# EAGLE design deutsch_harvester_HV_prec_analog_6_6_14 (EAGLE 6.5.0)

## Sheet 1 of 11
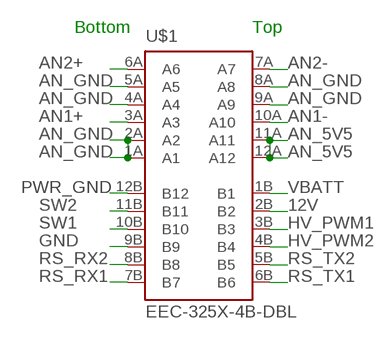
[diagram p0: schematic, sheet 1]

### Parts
U$1  EEC-325X-4B-DBL  [DEUTSCH_EEC_325X-4B]

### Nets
12V: U$1.2B(B2) ; also sheet 2
AN1+: U$1.3A(A3) ; also sheet 7
AN1-: U$1.10A(A10) ; also sheet 7
AN2+: U$1.6A(A6) ; also sheet 9
AN2-: U$1.7A(A7) ; also sheet 9
AN_5V5: U$1.11A(A11) U$1.12A(A12) ; also sheet 3,7,8,9
AN_GND: U$1.1A(A1) U$1.2A(A2) U$1.4A(A4) U$1.5A(A5) U$1.8A(A8) U$1.9A(A9) ; also sheet 7,8,9
GND: U$1.9B(B9) ; also sheet 2,3,4,5,6,8,10,11
HV_PWM1: U$1.3B(B3) ; also sheet 10
HV_PWM2: U$1.4B(B4) ; also sheet 10
PWR_GND: U$1.12B(B12) ; also sheet 2,10
RS_RX1: U$1.7B(B7) ; also sheet 5
RS_RX2: U$1.8B(B8) ; also sheet 5
RS_TX1: U$1.6B(B6) ; also sheet 5
RS_TX2: U$1.5B(B5) ; also sheet 5
SW1: U$1.10B(B10) ; also sheet 4
SW2: U$1.11B(B11) ; also sheet 4
VBATT: U$1.1B(B1) ; also sheet 2

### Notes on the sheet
- Bottom | Top

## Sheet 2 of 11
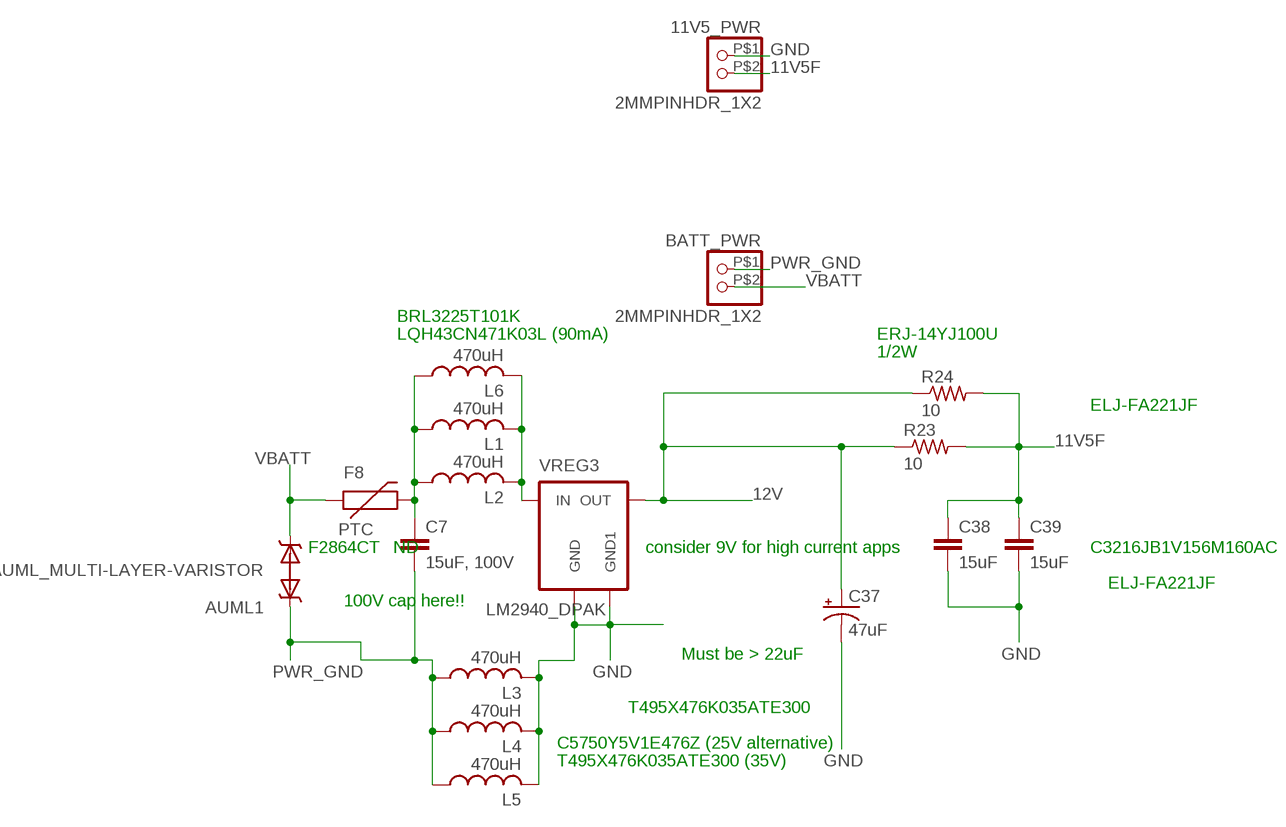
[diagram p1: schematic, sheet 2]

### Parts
11V5_PWR  2MMPINHDR_1X2  [2MMPINHDR_1X2]
AUML1  AUML_MULTI-LAYER-VARISTOR  [SMT_CAP_2220]
BATT_PWR  2MMPINHDR_1X2  [2MMPINHDR_1X2]
C7  15uF, 100V  C-EUC2220K  [C2220K]
C37  47uF  CPOL-USD/7343-31W  [D/7343-31W]
C38  15uF  C-EUC1206  [C1206]
C39  15uF  C-EUC1206  [C1206]
F8  PTC  [R_1206]
L1  470uH  L-USL1812  [L1812]
L2  470uH  L-USL1812  [L1812]
L3  470uH  L-USL1812  [L1812]
L4  470uH  L-USL1812  [L1812]
L5  470uH  L-USL1812  [L1812]
L6  470uH  L-USL1812  [L1812]
R23  10  R-US_R1210  [R1210]
R24  10  R-US_R1210  [R1210]
VREG3  LM2940_DPAK  [DPAK_TO263-3]

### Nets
11V5F: 11V5_PWR.P$2 C38.1 C39.1 R23.2 R24.2 ; also sheet 3
12V: C37.+ R23.1 R24.1 VREG3.3(OUT) ; also sheet 1
GND: 11V5_PWR.P$1 C37.- C38.2 C39.2 L3.2 L4.2 L5.2 VREG3.2(GND) VREG3.4(GND1) ; also sheet 1,3,4,5,6,8,10,11
N$1: C7.1 F8.2 L1.1 L2.1 L6.1
N$3: L1.2 L2.2 L6.2 VREG3.1(IN)
PWR_GND: AUML1.1 BATT_PWR.P$1 C7.2 L3.1 L4.1 L5.1 ; also sheet 1,10
VBATT: AUML1.2 BATT_PWR.P$2 F8.1 ; also sheet 1

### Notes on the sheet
- BRL3225T101K
- LQH43CN471K03L (90mA) | ERJ-14YJ100U
- 1/2W
- ELJ-FA221JF
- F2864CT‑ND | consider 9V for high current apps | C3216JB1V156M160AC
- ELJ-FA221JF
- 100V cap here!!
- Must be > 22uF
- T495X476K035ATE300
- C5750Y5V1E476Z (25V alternative)
- T495X476K035ATE300 (35V)

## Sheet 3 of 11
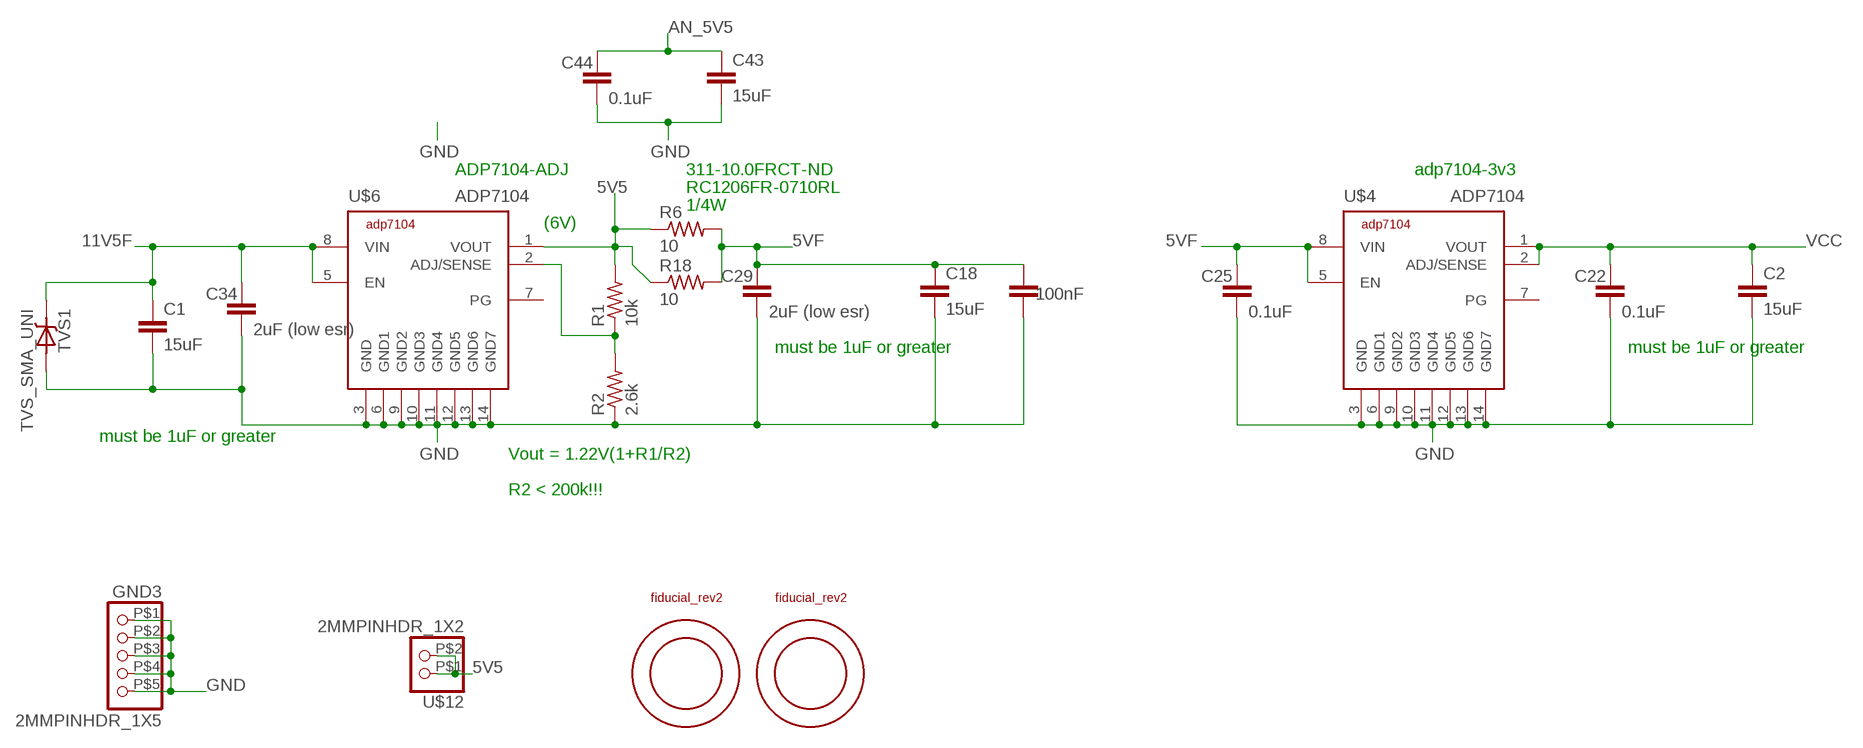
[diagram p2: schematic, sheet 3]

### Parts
C1  15uF  C-EUC1206  [C1206]
C2  15uF  C-EUC1206  [C1206]
C18  15uF  C-EUC1206  [C1206]
C22  0.1uF  C-EUC0805  [C0805]
C23  100nF  C-EUC0805  [C0805]
C25  0.1uF  C-EUC0805  [C0805]
C29  2uF (low esr)  C-EUC0805  [C0805]
C34  2uF (low esr)  C-EUC0805  [C0805]
C43  15uF  C-EUC1206  [C1206]
C44  0.1uF  C-EUC0805  [C0805]
GND3  2MMPINHDR_1X5  [2MMPINHDR_1X5]
R1  10k  R-US_R0805  [R0805]
R2  2.6k  R-US_R0805  [R0805]
R6  10  R-US_R1210  [R1210]
R18  10  R-US_R1210  [R1210]
TVS1  TVS_SMA_UNI  [DO-214AC(SMA)]
U$4  ADP7104  [SO8_GND_PAD]
U$6  ADP7104  [SO8_GND_PAD]
U$10  FIDUCIAL_REV2  [FIDUCIAL_REV2]
U$11  FIDUCIAL_REV2  [FIDUCIAL_REV2]
U$12  2MMPINHDR_1X2  [2MMPINHDR_1X2]

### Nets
5V5: R1.2 R6.1 R18.1 U$6.1(VOUT) U$12.P$1 U$12.P$2 ; also sheet 8
5VF: C18.1 C23.1 C25.1 C29.1 R6.2 R18.2 U$4.5(EN) U$4.8(VIN)
11V5F: C1.1 C34.1 TVS1.C U$6.5(EN) U$6.8(VIN) ; also sheet 2
AN_5V5: C43.1 C44.1 ; also sheet 1,7,8,9
GND: C1.2 C2.2 C18.2 C22.2 C23.2 C25.2 C29.2 C34.2 C43.2 C44.2 GND3.P$1 GND3.P$2 GND3.P$3 GND3.P$4 GND3.P$5 R2.1 TVS1.A U$4.3(GND) U$4.6(GND1) U$4.9(GND2) U$4.10(GND3) U$4.11(GND4) U$4.12(GND5) U$4.13(GND6) U$4.14(GND7) U$6.3(GND) U$6.6(GND1) U$6.9(GND2) U$6.10(GND3) U$6.11(GND4) U$6.12(GND5) U$6.13(GND6) U$6.14(GND7) ; also sheet 1,2,4,5,6,8,10,11
N$6: R1.1 R2.2 U$6.2(ADJ/SENSE)
VCC: C2.1 C22.1 U$4.1(VOUT) U$4.2(ADJ/SENSE) ; also sheet 4,5,6,11
Unconnected: U$4.7(PG) U$6.7(PG)

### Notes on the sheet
- ADP7104-ADJ | 311-10.0FRCT-ND | adp7104-3v3
- RC1206FR-0710RL
- 1/4W
- (6V)
- must be 1uF or greater | must be 1uF or greater
- must be 1uF or greater
- Vout = 1.22V(1+R1/R2)
- R2 < 200k!!!

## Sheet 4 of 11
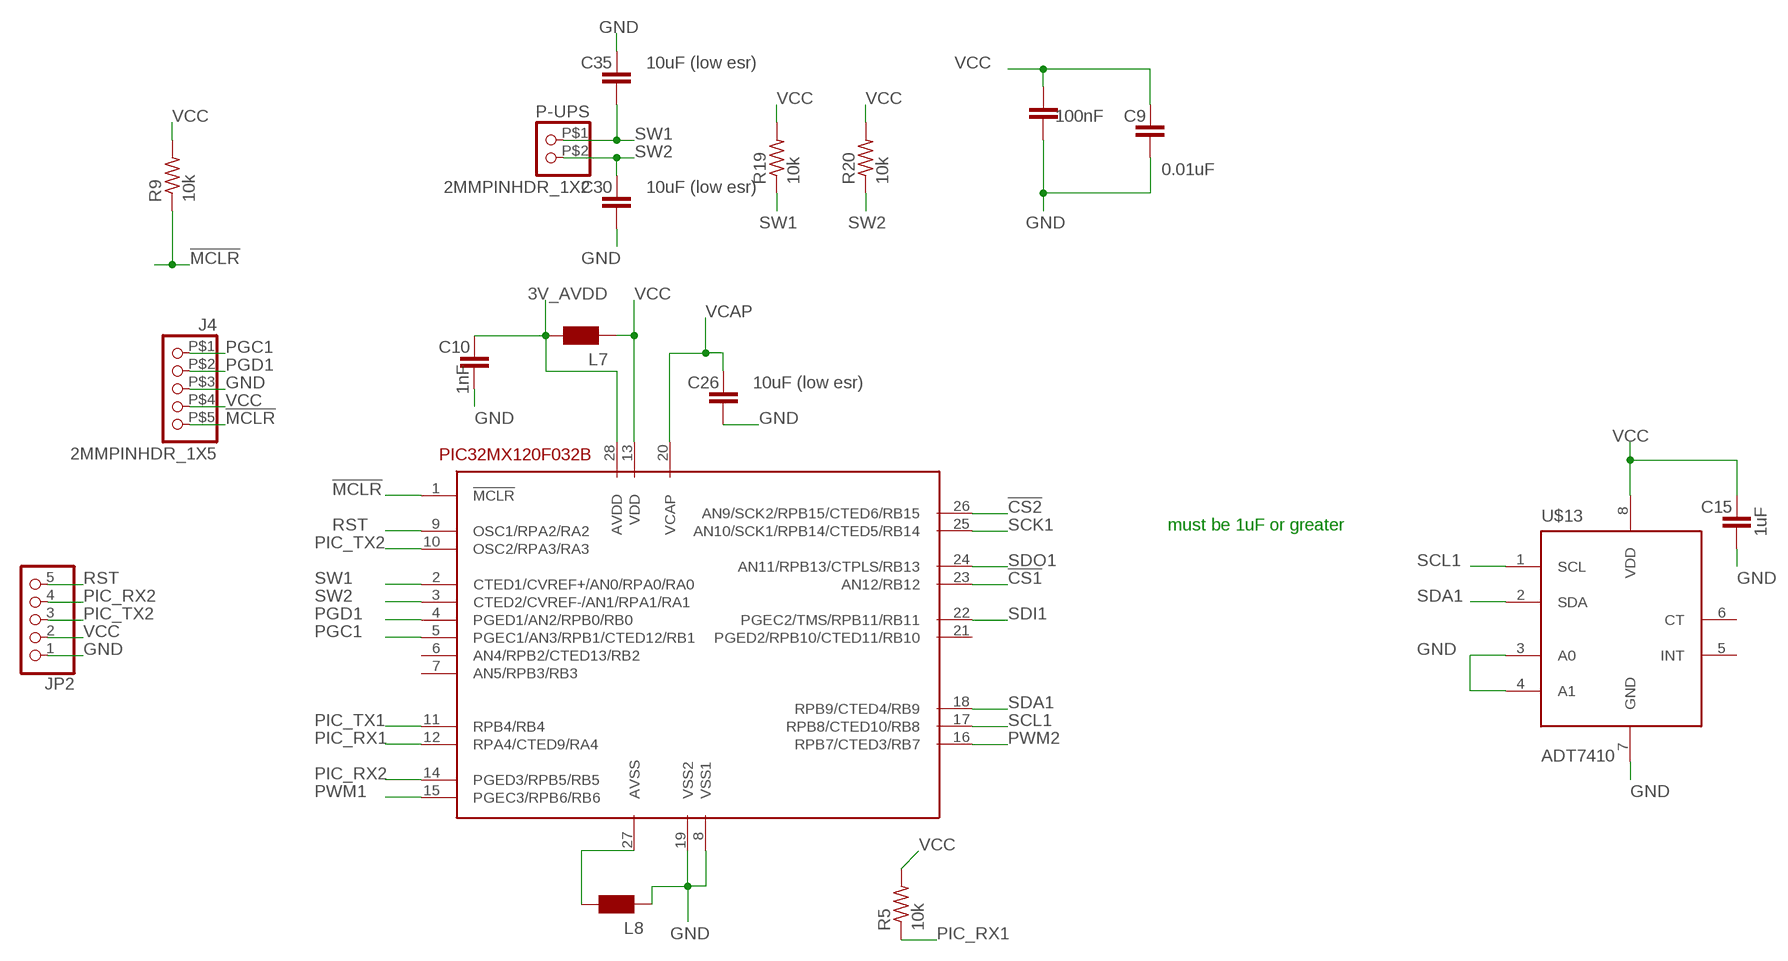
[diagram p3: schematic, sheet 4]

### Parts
C8  100nF  C-EUC0805  [C0805]
C9  0.01uF  C-EUC0805  [C0805]
C10  1nF  C-EUC0805  [C0805]
C15  1uF  C-EUC0805  [C0805]
C26  10uF (low esr)  C-EUC0805  [C0805]
C30  10uF (low esr)  C-EUC0805  [C0805]
C35  10uF (low esr)  C-EUC0805  [C0805]
J4  2MMPINHDR_1X5  [2MMPINHDR_1X5]
JP2  PINHD-1X5  [1X05]
L7  WE-CBF_1206  [1206]
L8  WE-CBF_1206  [1206]
P-UPS  2MMPINHDR_1X2  [2MMPINHDR_1X2]
R5  10k  R-US_R0805  [R0805]
R9  10k  R-US_R0805  [R0805]
R19  10k  R-US_R0805  [R0805]
R20  10k  R-US_R0805  [R0805]
U2  PIC32MX120F032B-28SOIC  [SOICW28_MICROCHIP]
U$13  ADT7410  [SO8]

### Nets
3V_AVDD: C10.1 L7.2 U2.28(AVDD)
!CS1: U2.23(AN12/RB12) ; also sheet 7
!CS2: U2.26(AN9/SCK2/RPB15/CTED6/RB15) ; also sheet 9
!MCLR: J4.P$5 R9.1 U2.1(!MCLR)
GND: C8.2 C9.2 C10.2 C15.2 C26.2 C30.2 C35.1 J4.P$3 JP2.1 L8.1 U2.8(VSS1) U2.19(VSS2) U$13.3(A0) U$13.4(A1) U$13.7(GND) ; also sheet 1,2,3,5,6,8,10,11
N$8: L8.2 U2.27(AVSS)
PGC1: J4.P$1 U2.5(PGEC1/AN3/RPB1/CTED12/RB1)
PGD1: J4.P$2 U2.4(PGED1/AN2/RPB0/RB0)
PIC_RX1: R5.1 U2.12(RPA4/CTED9/RA4) ; also sheet 5
PIC_RX2: JP2.4 U2.14(PGED3/RPB5/RB5) ; also sheet 5
PIC_TX1: U2.11(RPB4/RB4) ; also sheet 5
PIC_TX2: JP2.3 U2.10(OSC2/RPA3/RA3) ; also sheet 5
PWM1: U2.15(PGEC3/RPB6/RB6) ; also sheet 10
PWM2: U2.16(RPB7/CTED3/RB7) ; also sheet 10
RST: JP2.5 U2.9(OSC1/RPA2/RA2)
SCK1: U2.25(AN10/SCK1/RPB14/CTED5/RB14) ; also sheet 7,9
SCL1: U2.17(RPB8/CTED10/RB8) U$13.1(SCL) ; also sheet 6,11
SDA1: U2.18(RPB9/CTED4/RB9) U$13.2(SDA) ; also sheet 6,11
SDI1: U2.22(PGEC2/TMS/RPB11/RB11) ; also sheet 7,9
SDO1: U2.24(AN11/RPB13/CTPLS/RB13)
SW1: C35.2 P-UPS.P$1 R19.1 U2.2(CTED1/CVREF+/AN0/RPA0/RA0) ; also sheet 1
SW2: C30.1 P-UPS.P$2 R20.1 U2.3(CTED2/CVREF-/AN1/RPA1/RA1) ; also sheet 1
VCAP: C26.1 U2.20(VCAP)
VCC: C8.1 C9.1 C15.1 J4.P$4 JP2.2 L7.1 R5.2 R9.2 R19.2 R20.2 U2.13(VDD) U$13.8(VDD) ; also sheet 3,5,6,11
Unconnected: U2.6(AN4/RPB2/CTED13/RB2) U2.7(AN5/RPB3/RB3) U2.21(PGED2/RPB10/CTED11/RB10) U$13.5(INT) U$13.6(CT)

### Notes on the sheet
- must be 1uF or greater

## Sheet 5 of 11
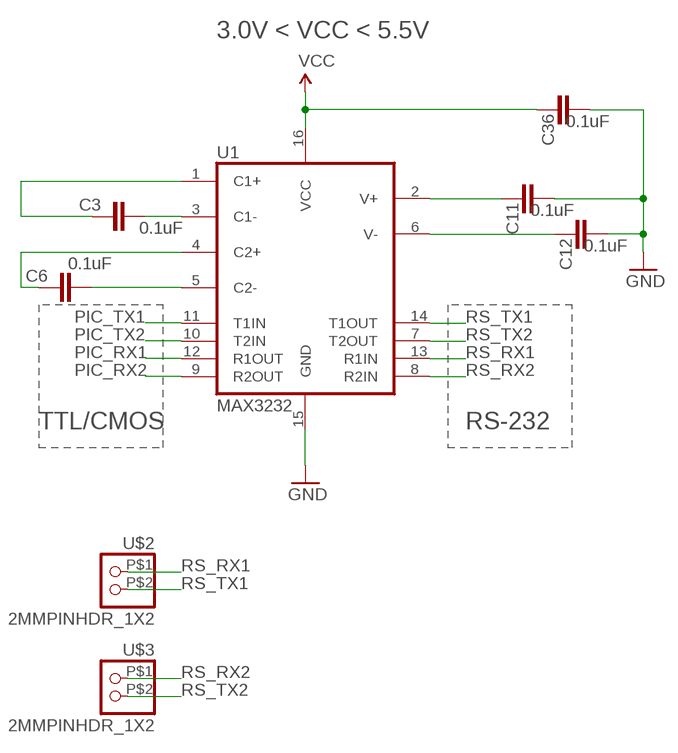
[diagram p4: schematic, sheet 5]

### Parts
C3  0.1uF  C-EUC0805  [C0805]
C6  0.1uF  C-EUC0805  [C0805]
C11  0.1uF  C-EUC0805  [C0805]
C12  0.1uF  C-EUC0805  [C0805]
C36  0.1uF  C-EUC0805  [C0805]
U1  MAX3232  MAX232SOIC16  [SO016]
U$2  2MMPINHDR_1X2  [2MMPINHDR_1X2]
U$3  2MMPINHDR_1X2  [2MMPINHDR_1X2]

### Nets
C1+: C3.1 U1.1(C1+)
C1-: C3.2 U1.3(C1-)
C2+: C6.1 U1.4(C2+)
C2-: C6.2 U1.5(C2-)
GND: C11.2 C12.2 C36.2 U1.15(GND) ; also sheet 1,2,3,4,6,8,10,11
PIC_RX1: U1.12(R1OUT) ; also sheet 4
PIC_RX2: U1.9(R2OUT) ; also sheet 4
PIC_TX1: U1.11(T1IN) ; also sheet 4
PIC_TX2: U1.10(T2IN) ; also sheet 4
RS_RX1: U1.13(R1IN) U$2.P$1 ; also sheet 1
RS_RX2: U1.8(R2IN) U$3.P$1 ; also sheet 1
RS_TX1: U1.14(T1OUT) U$2.P$2 ; also sheet 1
RS_TX2: U1.7(T2OUT) U$3.P$2 ; also sheet 1
V+: C11.1 U1.2(V+)
V-: C12.1 U1.6(V-)
VCC: C36.1 U1.16(VCC) ; also sheet 3,4,6,11

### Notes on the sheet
- 3.0V < VCC < 5.5V
- TTL/CMOS | RS-232

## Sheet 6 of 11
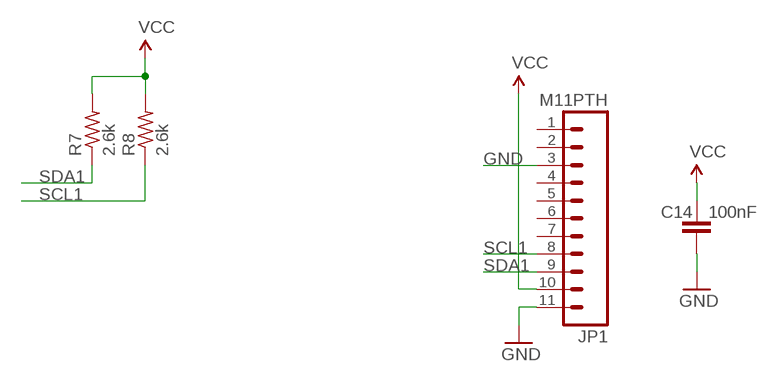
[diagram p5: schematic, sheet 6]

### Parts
C14  100nF  C-EUC0805  [C0805]
JP1  M11PTH  [1X11]
R7  2.6k  R-US_R0805  [R0805]
R8  2.6k  R-US_R0805  [R0805]

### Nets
GND: C14.2 JP1.3 JP1.11 ; also sheet 1,2,3,4,5,8,10,11
SCL1: JP1.8 R8.1 ; also sheet 4,11
SDA1: JP1.9 R7.1 ; also sheet 4,11
VCC: C14.1 JP1.10 R7.2 R8.2 ; also sheet 3,4,5,11
Unconnected: JP1.1 JP1.2 JP1.4 JP1.5 JP1.6 JP1.7

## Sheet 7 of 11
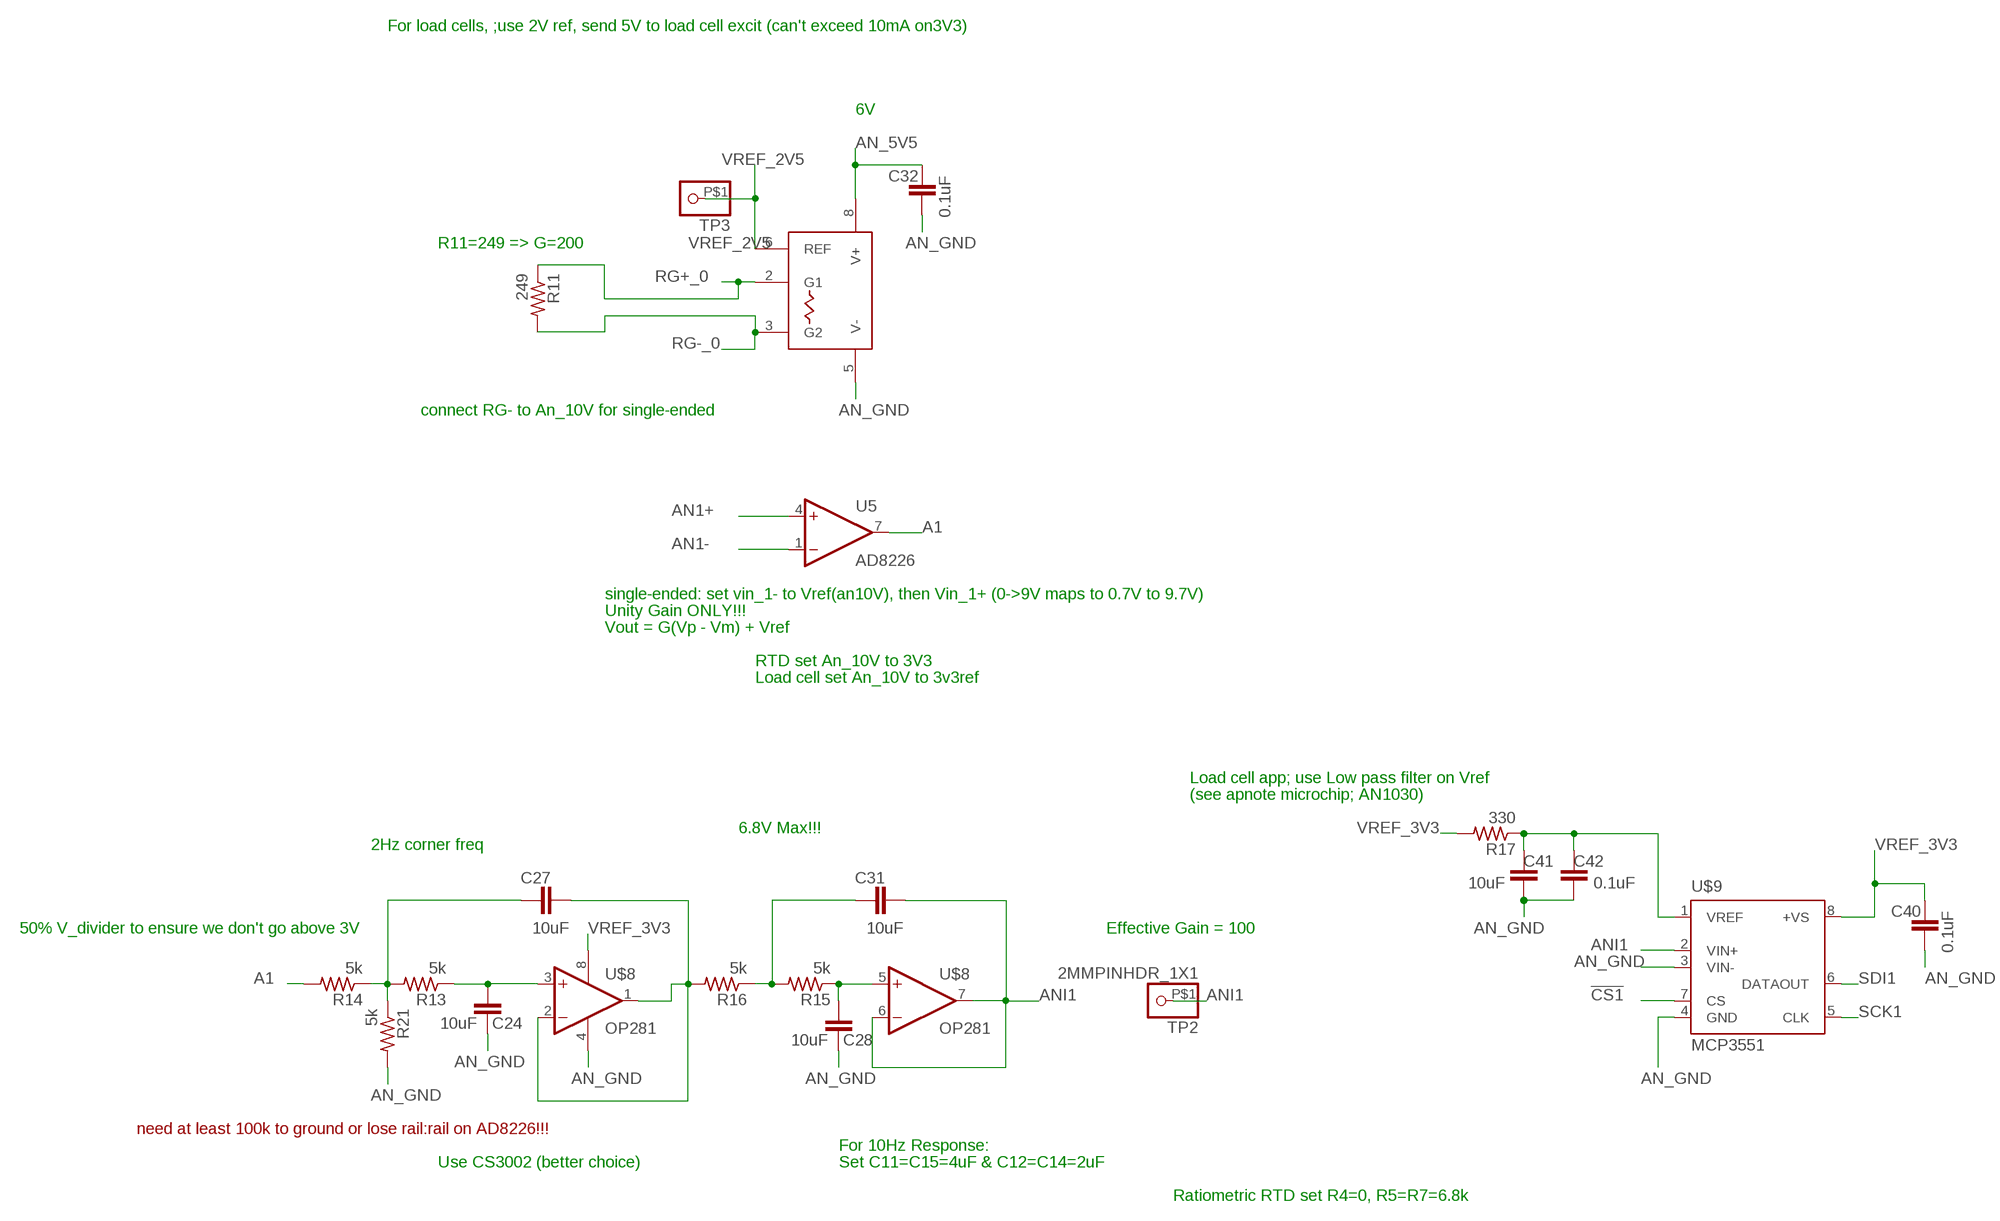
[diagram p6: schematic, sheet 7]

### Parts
C24  10uF  C-EUC0805  [C0805]
C27  10uF  C-EUC0805  [C0805]
C28  10uF  C-EUC0805  [C0805]
C31  10uF  C-EUC0805  [C0805]
C32  0.1uF  C-EUC0805  [C0805]
C40  0.1uF  C-EUC0805  [C0805]
C41  10uF  C-EUC0805  [C0805]
C42  0.1uF  C-EUC0805  [C0805]
R11  249  R-US_R0805  [R0805]
R13  5k  R-US_R0805  [R0805]
R14  5k  R-US_R0805  [R0805]
R15  5k  R-US_R0805  [R0805]
R16  5k  R-US_R0805  [R0805]
R17  330  R-US_R0805  [R0805]
R21  5k  R-US_R0805  [R0805]
TP2  2MMPINHDR_1X1  [2MMPINHDR_1X1]
TP3  2MMPINHDR_1X1  [2MMPINHDR_1X1]
U5  AD8226  [SO8@1]
U$8  OP281  [SO_08]
U$9  MCP3551  [SO_08]

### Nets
!CS1: U$9.7(CS) ; also sheet 4
A1: R14.2 U5.7(OUT)
AN1+: U5.4(+IN) ; also sheet 1
AN1-: U5.1(-IN) ; also sheet 1
AN_5V5: C32.1 U5.8(V+) ; also sheet 1,3,8,9
AN_GND: C24.1 C28.1 C32.2 C40.2 C41.1 C42.1 R21.2 U5.5(V-) U$8.4(V-) U$9.3(VIN-) U$9.4(GND) ; also sheet 1,8,9
ANI1: C31.1 TP2.P$1 U$8.6(-IN2) U$8.7(OUT2) U$9.2(VIN+)
N$2: C24.2 R13.1 U$8.3(+IN1)
N$4: C27.1 R16.2 U$8.1(OUT1) U$8.2(-IN1)
N$5: C27.2 R13.2 R14.1 R21.1
N$9: C41.2 C42.2 R17.1 U$9.1(VREF)
N$13: C31.2 R15.2 R16.1
N$14: C28.2 R15.1 U$8.5(+IN2)
RG+_0: R11.1 U5.2(G1)
RG-_0: R11.2 U5.3(G2)
SCK1: U$9.5(CLK) ; also sheet 4,9
SDI1: U$9.6(DATAOUT) ; also sheet 4,9
VREF_2V5: TP3.P$1 U5.6(REF) ; also sheet 8,9
VREF_3V3: C40.1 R17.2 U$8.8(V+) U$9.8(+VS) ; also sheet 8,9

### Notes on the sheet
- For load cells, ;use 2V ref, send 5V to load cell excit (can't exceed 10mA on3V3)
- 6V
- R11=249 => G=200
- connect RG- to An_10V for single-ended
- single-ended: set vin_1- to Vref(an10V), then Vin_1+ (0->9V maps to 0.7V to 9.7V)
- Unity Gain ONLY!!!
- Vout = G(Vp - Vm) + Vref
- RTD set An_10V to 3V3
- Load cell set An_10V to 3v3ref
- Load cell app; use Low pass filter on Vref
- (see apnote microchip; AN1030)
- 6.8V Max!!!
- 2Hz corner freq
- 50% V_divider to ensure we don't go above 3V | Effective Gain = 100
- need at least 100k to ground or lose rail:rail on AD8226!!!
- For 10Hz Response:
- Use CS3002 (better choice) | Set C11=C15=4uF & C12=C14=2uF
- Ratiometric RTD set R4=0, R5=R7=6.8k

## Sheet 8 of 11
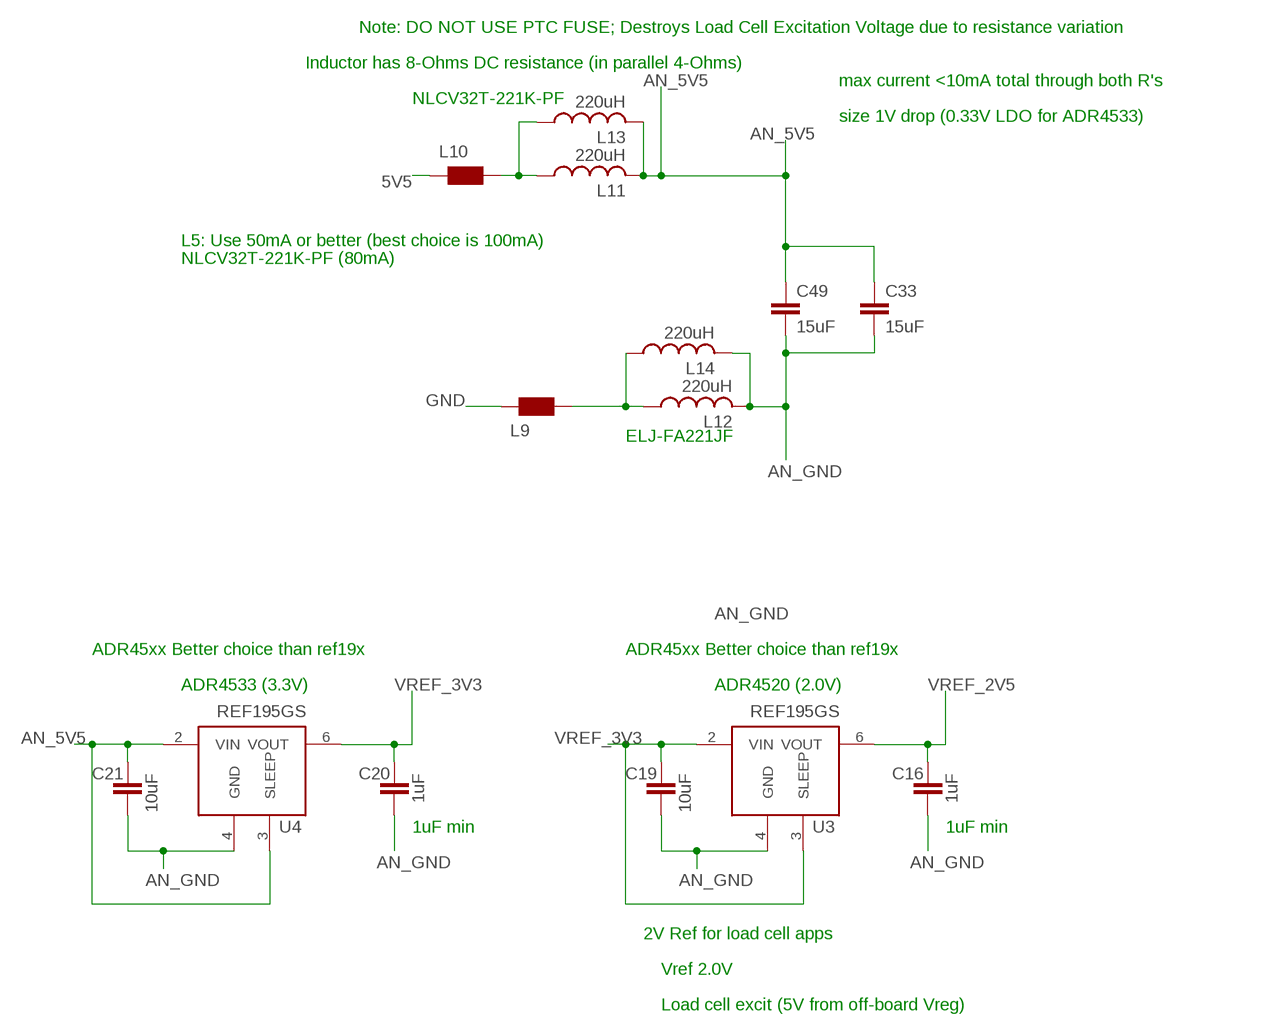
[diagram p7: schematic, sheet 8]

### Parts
C16  1uF  C-EUC0805  [C0805]
C19  10uF  C-EUC0805  [C0805]
C20  1uF  C-EUC0805  [C0805]
C21  10uF  C-EUC0805  [C0805]
C33  15uF  C-EUC1206  [C1206]
C49  15uF  C-EUC1206  [C1206]
L9  WE-CBF_1206  [1206]
L10  WE-CBF_1206  [1206]
L11  220uH  L-USL3225P  [L3225P]
L12  220uH  L-USL3225P  [L3225P]
L13  220uH  L-USL3225P  [L3225P]
L14  220uH  L-USL3225P  [L3225P]
U3  REF195GS  [SO8@1]
U4  REF195GS  [SO8@1]

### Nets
5V5: L10.1 ; also sheet 3
AN_5V5: C21.1 C33.1 C49.1 L11.2 L13.2 U4.2(VIN) U4.3(SLEEP) ; also sheet 1,3,7,9
AN_GND: C16.2 C19.2 C20.2 C21.2 C33.2 C49.2 L12.2 L14.2 U3.4(GND) U4.4(GND) ; also sheet 1,7,9
GND: L9.1 ; also sheet 1,2,3,4,5,6,10,11
N$7: L10.2 L11.1 L13.1
PWR_GND1: L9.2 L12.1 L14.1
VREF_2V5: C16.1 U3.6(VOUT) ; also sheet 7,9
VREF_3V3: C19.1 C20.1 U3.2(VIN) U3.3(SLEEP) U4.6(VOUT) ; also sheet 7,9

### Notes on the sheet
- Note: DO NOT USE PTC FUSE; Destroys Load Cell Excitation Voltage due to resistance variation
- Inductor has 8-Ohms DC resistance (in parallel 4-Ohms)
- max current <10mA total through both R's
- NLCV32T-221K-PF
- size 1V drop (0.33V LDO for ADR4533)
- L5: Use 50mA or better (best choice is 100mA)
- NLCV32T-221K-PF (80mA)
- ELJ-FA221JF
- ADR45xx Better choice than ref19x | ADR45xx Better choice than ref19x
- ADR4533 (3.3V) | ADR4520 (2.0V)
- 1uF min | 1uF min
- 2V Ref for load cell apps
- Vref 2.0V
- Load cell excit (5V from off-board Vreg)

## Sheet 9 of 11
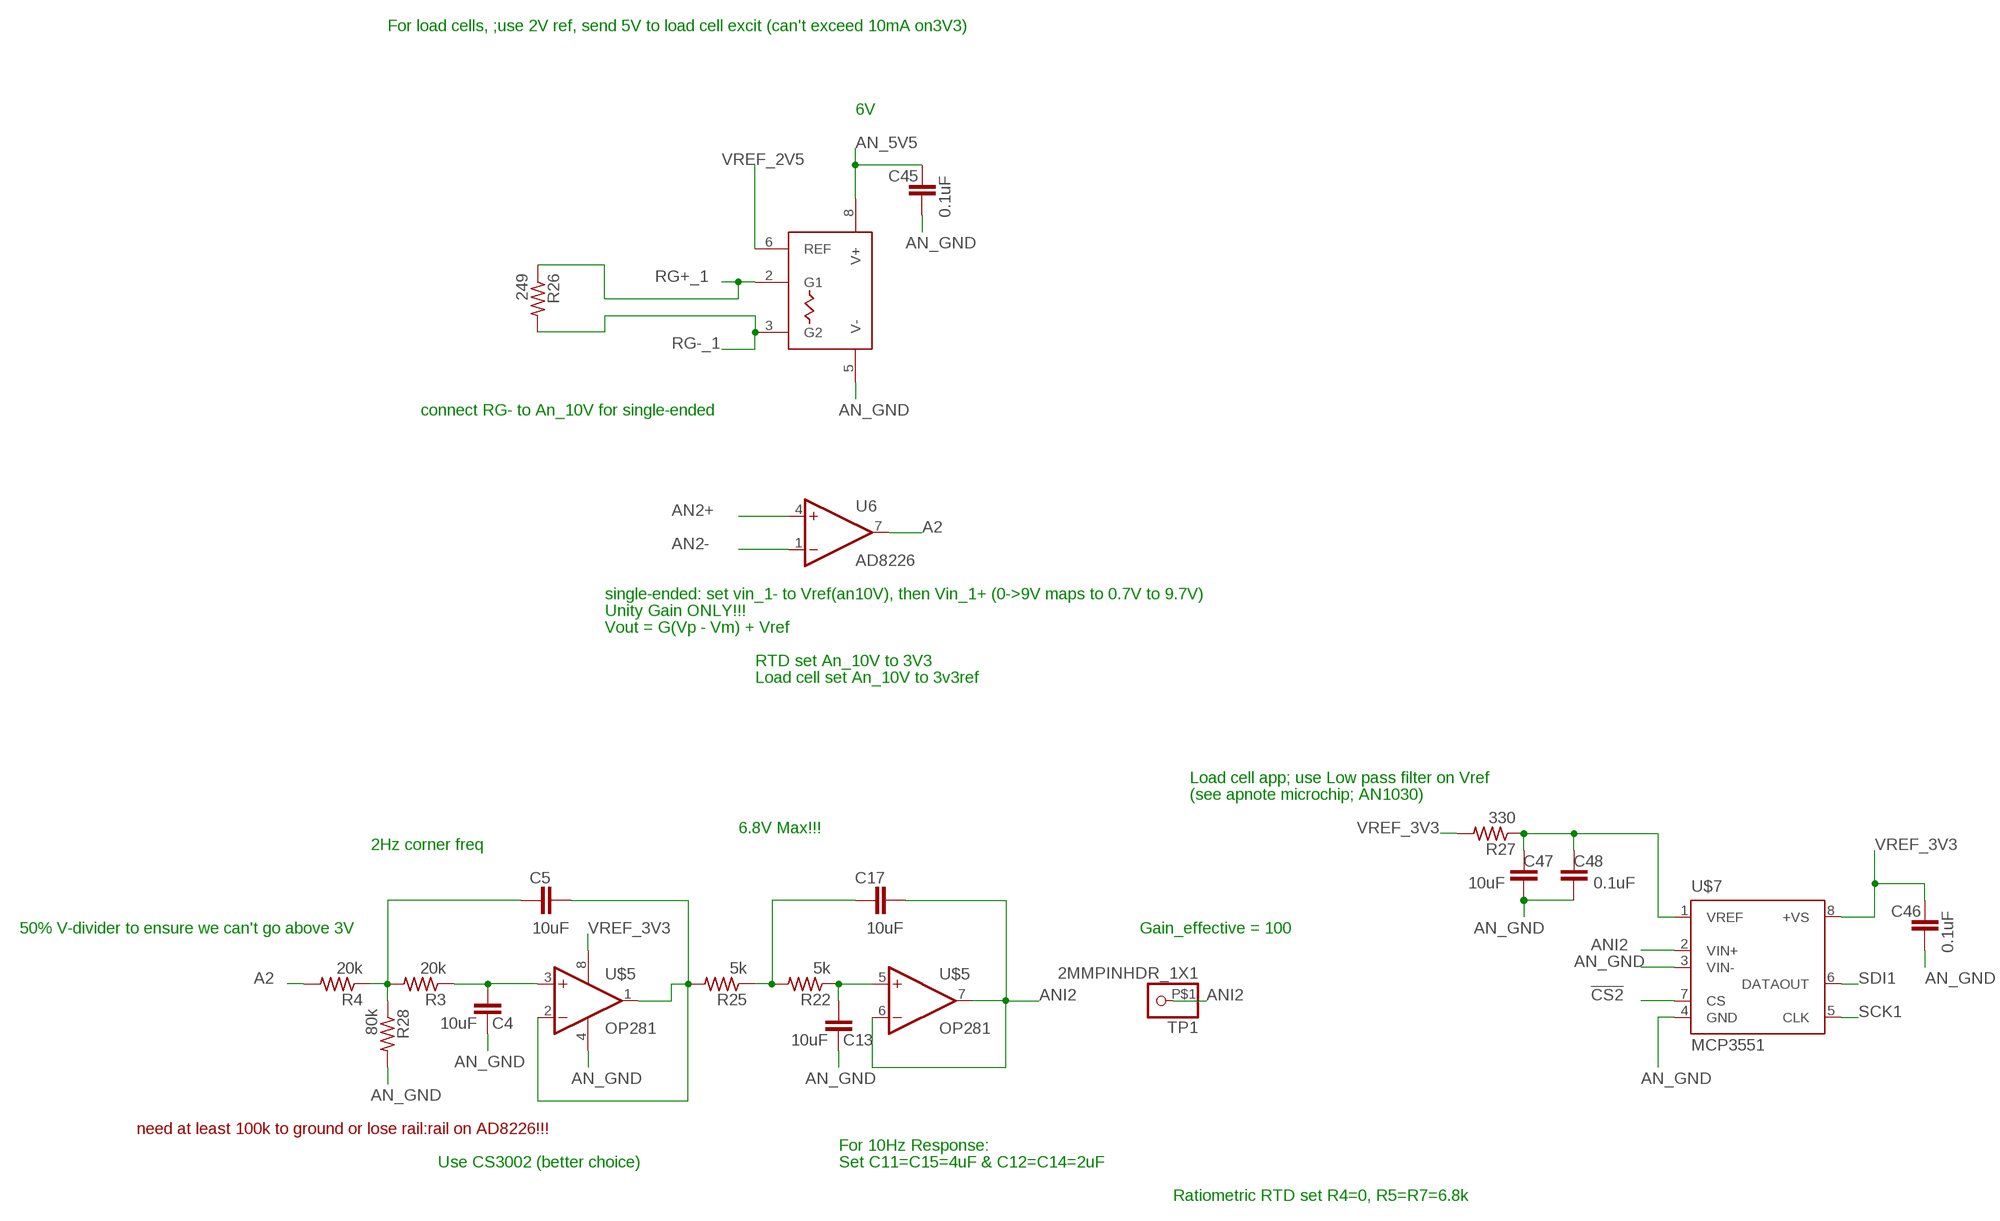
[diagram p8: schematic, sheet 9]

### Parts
C4  10uF  C-EUC0805  [C0805]
C5  10uF  C-EUC0805  [C0805]
C13  10uF  C-EUC0805  [C0805]
C17  10uF  C-EUC0805  [C0805]
C45  0.1uF  C-EUC0805  [C0805]
C46  0.1uF  C-EUC0805  [C0805]
C47  10uF  C-EUC0805  [C0805]
C48  0.1uF  C-EUC0805  [C0805]
R3  20k  R-US_R0805  [R0805]
R4  20k  R-US_R0805  [R0805]
R22  5k  R-US_R0805  [R0805]
R25  5k  R-US_R0805  [R0805]
R26  249  R-US_R0805  [R0805]
R27  330  R-US_R0805  [R0805]
R28  80k  R-US_R0805  [R0805]
TP1  2MMPINHDR_1X1  [2MMPINHDR_1X1]
U6  AD8226  [SO8@1]
U$5  OP281  [SO_08]
U$7  MCP3551  [SO_08]

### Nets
!CS2: U$7.7(CS) ; also sheet 4
A2: R4.2 U6.7(OUT)
AN2+: U6.4(+IN) ; also sheet 1
AN2-: U6.1(-IN) ; also sheet 1
AN_5V5: C45.1 U6.8(V+) ; also sheet 1,3,7,8
AN_GND: C4.1 C13.1 C45.2 C46.2 C47.1 C48.1 R28.2 U6.5(V-) U$5.4(V-) U$7.3(VIN-) U$7.4(GND) ; also sheet 1,7,8
ANI2: C17.1 TP1.P$1 U$5.6(-IN2) U$5.7(OUT2) U$7.2(VIN+)
N$15: C4.2 R3.1 U$5.3(+IN1)
N$16: C5.2 R3.2 R4.1 R28.1
N$17: C17.2 R22.2 R25.1
N$18: C13.2 R22.1 U$5.5(+IN2)
N$19: C5.1 R25.2 U$5.1(OUT1) U$5.2(-IN1)
N$20: C47.2 C48.2 R27.1 U$7.1(VREF)
RG+_1: R26.1 U6.2(G1)
RG-_1: R26.2 U6.3(G2)
SCK1: U$7.5(CLK) ; also sheet 4,7
SDI1: U$7.6(DATAOUT) ; also sheet 4,7
VREF_2V5: U6.6(REF) ; also sheet 7,8
VREF_3V3: C46.1 R27.2 U$5.8(V+) U$7.8(+VS) ; also sheet 7,8

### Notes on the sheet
- For load cells, ;use 2V ref, send 5V to load cell excit (can't exceed 10mA on3V3)
- 6V
- connect RG- to An_10V for single-ended
- single-ended: set vin_1- to Vref(an10V), then Vin_1+ (0->9V maps to 0.7V to 9.7V)
- Unity Gain ONLY!!!
- Vout = G(Vp - Vm) + Vref
- RTD set An_10V to 3V3
- Load cell set An_10V to 3v3ref
- Load cell app; use Low pass filter on Vref
- (see apnote microchip; AN1030)
- 6.8V Max!!!
- 2Hz corner freq
- 50% V-divider to ensure we can't go above 3V | Gain_effective = 100
- need at least 100k to ground or lose rail:rail on AD8226!!!
- For 10Hz Response:
- Use CS3002 (better choice) | Set C11=C15=4uF & C12=C14=2uF
- Ratiometric RTD set R4=0, R5=R7=6.8k

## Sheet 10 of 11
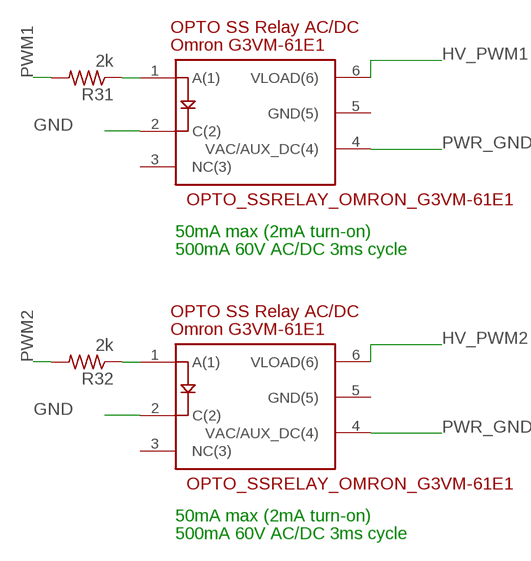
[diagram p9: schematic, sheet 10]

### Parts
R31  2k  R-US_R0805  [R0805]
R32  2k  R-US_R0805  [R0805]
U$43  OPTO_SSRELAY_OMRON_G3VM-61E1  [6-SMD_OMRON_SSRELAY]
U$44  OPTO_SSRELAY_OMRON_G3VM-61E1  [6-SMD_OMRON_SSRELAY]

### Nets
GND: U$43.2(C(2)) U$44.2(C(2)) ; also sheet 1,2,3,4,5,6,8,11
HV_PWM1: U$44.6(VLOAD(6)) ; also sheet 1
HV_PWM2: U$43.6(VLOAD(6)) ; also sheet 1
N$22: R31.1 U$44.1(A(1))
N$23: R32.1 U$43.1(A(1))
PWM1: R31.2 ; also sheet 4
PWM2: R32.2 ; also sheet 4
PWR_GND: U$43.4(VAC/AUX_DC(4)) U$44.4(VAC/AUX_DC(4)) ; also sheet 1,2
Unconnected: U$43.3(NC(3)) U$43.5(GND(5)) U$44.3(NC(3)) U$44.5(GND(5))

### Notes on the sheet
- 50mA max (2mA turn-on)
- 500mA 60V AC/DC 3ms cycle
- 50mA max (2mA turn-on)
- 500mA 60V AC/DC 3ms cycle

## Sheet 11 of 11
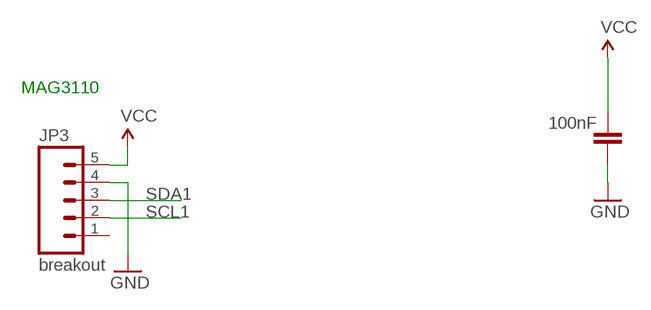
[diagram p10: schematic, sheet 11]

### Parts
C51  100nF  C-EUC0805  [C0805]
JP3  breakout  M05PTH  [1X05]

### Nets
GND: C51.2 JP3.4 ; also sheet 1,2,3,4,5,6,8,10
SCL1: JP3.2 ; also sheet 4,6
SDA1: JP3.3 ; also sheet 4,6
VCC: C51.1 JP3.5 ; also sheet 3,4,5,6
Unconnected: JP3.1

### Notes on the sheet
- MAG3110

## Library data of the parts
11V5_PWR BATT_PWR P-UPS = smd-special_28PIN_PIC32_11_3_2011:2MMPINHDR_1X2
AUML1 = smd-special_28PIN_PIC32_11_3_2011_MOD5_20_13:AUML_MULTI-LAYER-VARISTOR: V18AUMLA2220: 18V cont, 24.5V (5min. jump starts), 25Joule load dump, 40V max Clamp voltage
C1-C36 C38-C49 C51 = rcl:C-EU: CAPACITOR, European symbol
C37 = rcl:CPOL-US: POLARIZED CAPACITOR, American symbol
F8 = smd-special_28PIN_PIC32_11_3_2011_MOD4_1_13:PTC: Little Fuse: 1206L025YR, 16V, 250mA hold, 500mA trip Resetable Fuse
GND3 J4 = smd-special_28PIN_PIC32_11_3_2011_MOD5_20_13:2MMPINHDR_1X5
JP1 = SparkFun-Connectors:M11: Header 11 Standard 11-pin 0.1" header. Use with straight break away headers (SKU : PRT-00116), right angle break away headers (PRT-00553), swiss pins (PRT-00743), machine pins (PRT-00117), and female headers (PRT-00115).
JP2 = pinhead:PINHD-1X5: PIN HEADER
JP3 = SparkFun:M05: Header 5 Standard 5-pin 0.1" header. Use with straight break away headers (SKU : PRT-00116), right angle break away headers (PRT-00553), swiss pins (PRT-00743), machine pins (PRT-00117), and female headers (PRT-00115). Molex polarized connector foot print use with SKU : PRT-08230 with associated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
L1-L6 L11-L14 = rcl:L-US: INDUCTOR, American symbol
L7-L10 = wuerth-elektronik:WE-CBF: SMD EMI Suppression Ferrite Beads
R1-R9 R11 R13-R28 R31 R32 = rcl:R-US_: RESISTOR, American symbol
TP1-TP3 = smd-special_28PIN_PIC32_11_3_2011:2MMPINHDR_1X1
TVS1 = smd-special_28PIN_PIC32_11_3_2011_MOD5_20_13:TVS_SMA_UNI: SMAJ6.0A Uni-directional TVS 6V
U1 = SparkFun-DigitalIC:MAX232: RS232 Transceiver Very common IC. This is generically called 'MAX232', but works with the 3V equivalent MAX3232 generic ICs. Field tested and mother approved. Spark Fun Electronics SKU : COM-00316 (DIP) and COM-00589 (SMD); PROD_ID: IC-08171
U2 = smd-special_28PIN_PIC32_11_3_2011:PIC32MX120F032B-28SOIC
U3 U4 = analog-devices:REF195*: Precision Micropower, Low Dropout, Voltage References Low Supply Current: 45 mikroA max High Output Current: 30 mA Short Circuit Protection
U5 U6 = analog-devices:AD8226: Instrumentation Amp with Over-voltage protection
U$1 = smd-special_28PIN_PIC32_11_3_2011_MOD5_20_13:EEC-325X-4B-DBL
U$2 U$3 U$12 = smd-special_28PIN_PIC32_11_3_2011_MOD5_20_13:2MMPINHDR_1X2
U$4 U$6 = analog-devices:ADP7104: ADP7104 Low Noise LDO Voltage Regulator 15uV noise, 500mA source current
U$5 U$8 = smd-special_28PIN_PIC32_11_3_2011:OP281
U$7 U$9 = smd-special_28PIN_PIC32_11_3_2011:MCP3551
U$10 U$11 = smd-special:FIDUCIAL_REV2
U$13 = analog-devices:ADT7410: Precision I2C Temp Sensor
U$43 U$44 = SparkFun:OPTO_SSRELAY_OMRON_G3VM-61E1
VREG3 = smd-special_28PIN_PIC32_11_3_2011:LM2940_DPAK: lm2940 smt

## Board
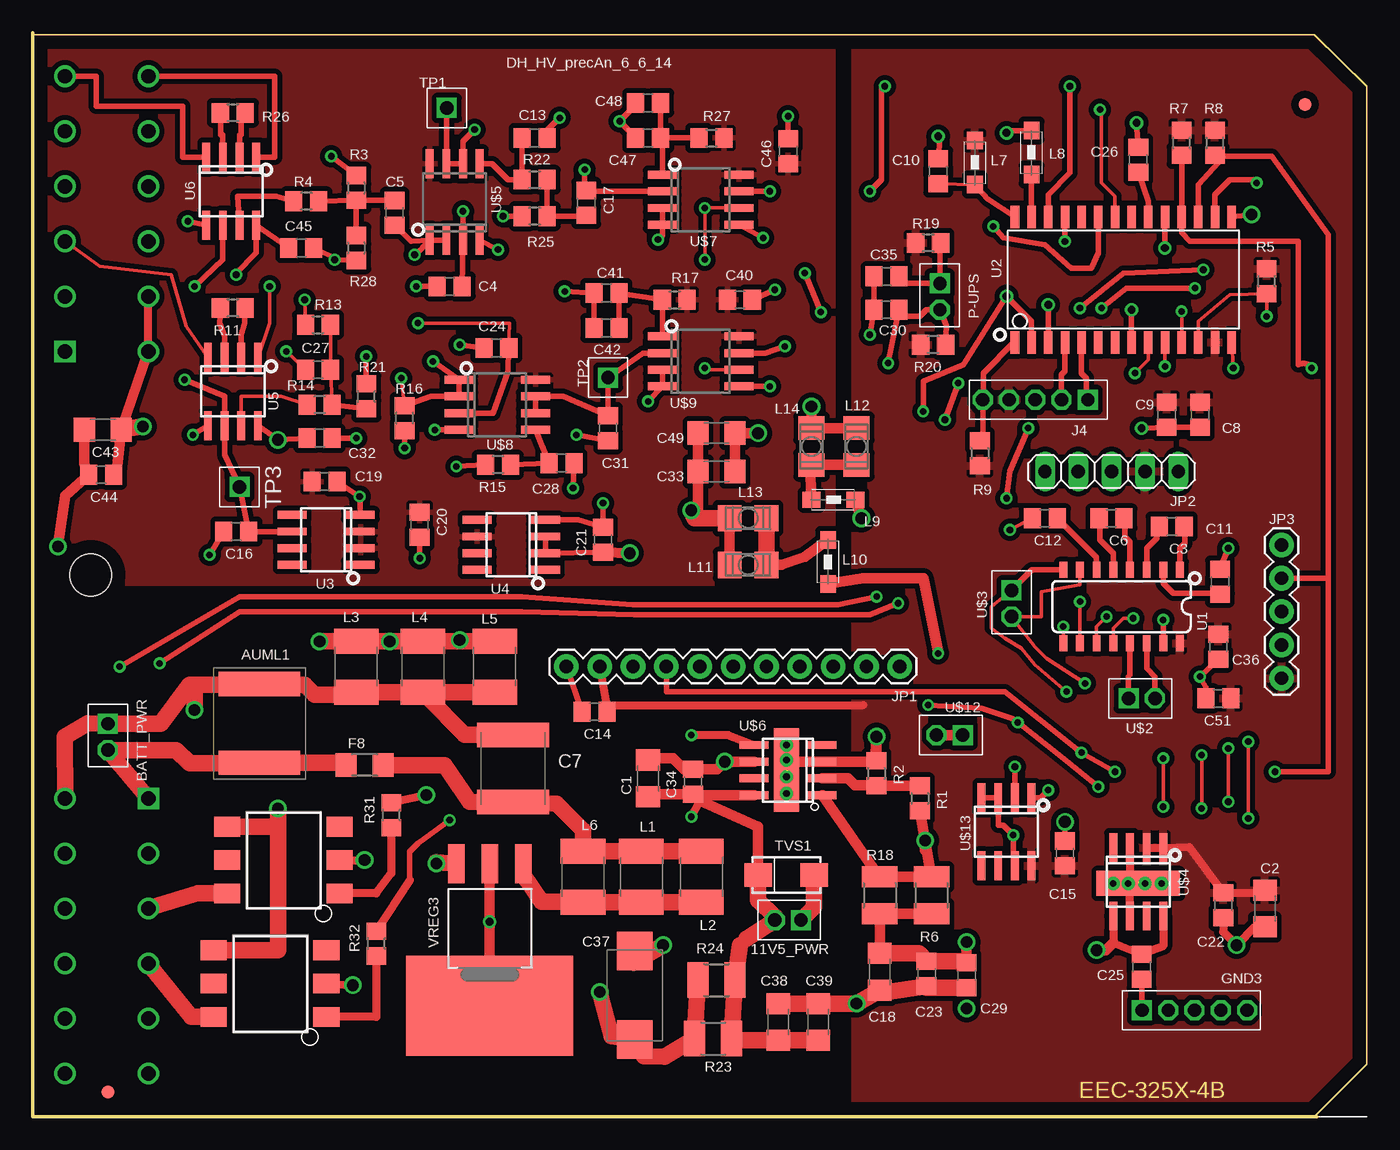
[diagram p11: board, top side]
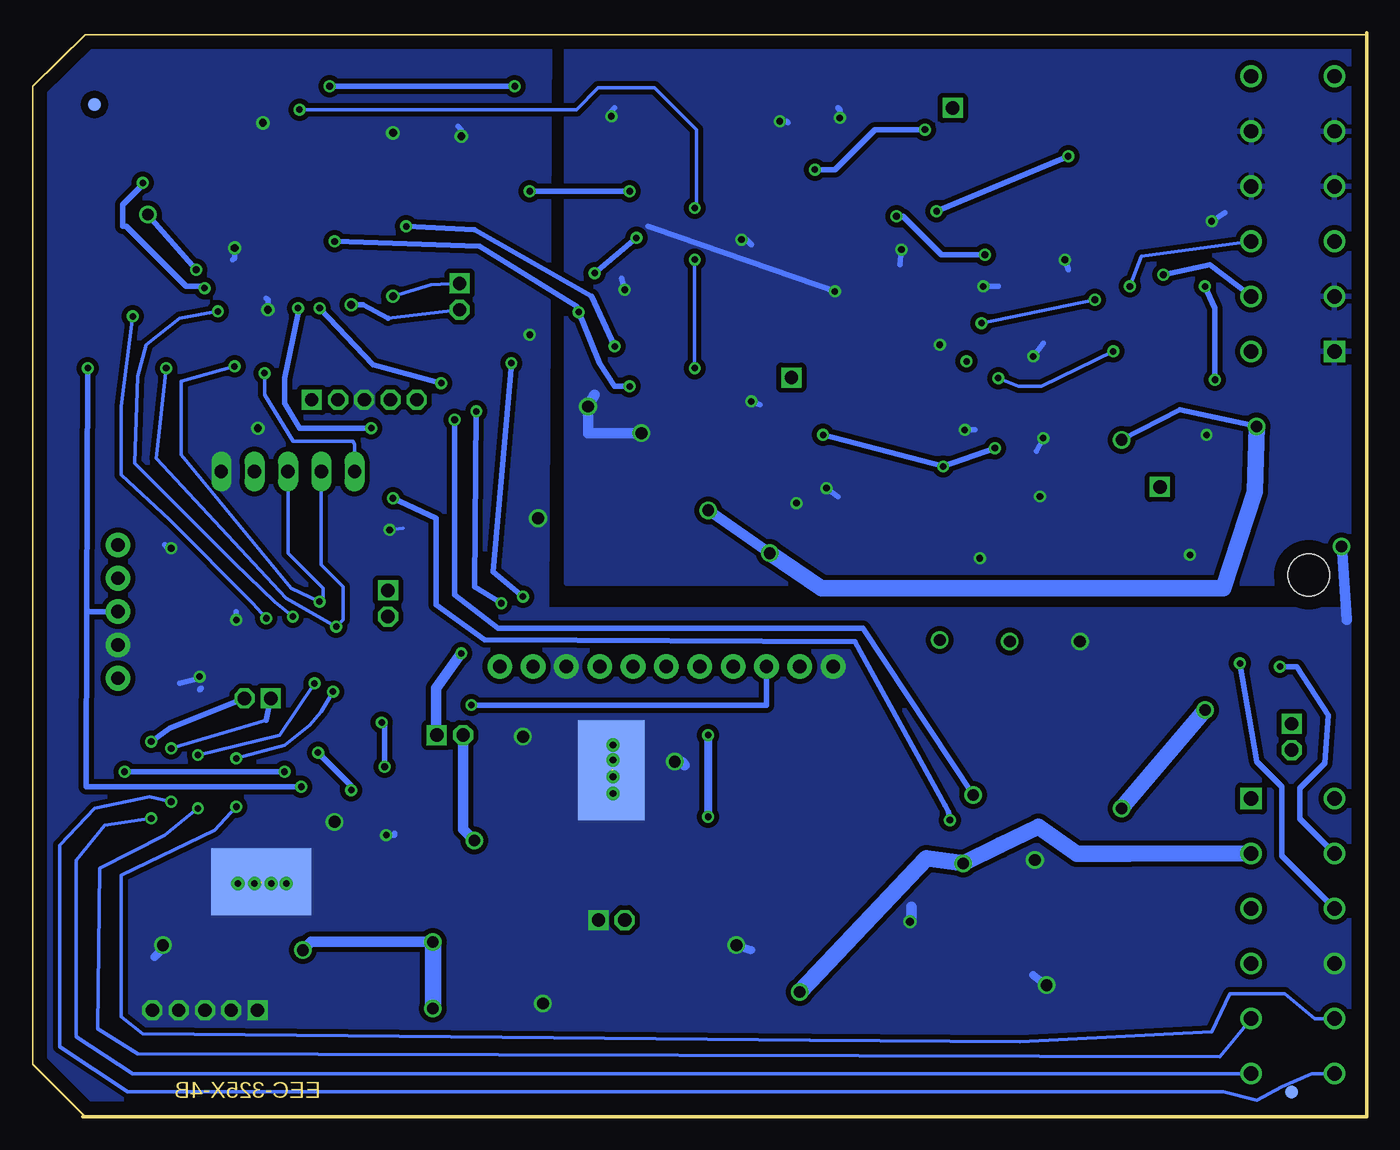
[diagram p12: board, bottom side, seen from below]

Size 101.6 x 82.55 mm. Coordinates in mm from the lower left corner, seen from the top.
Outline: 0,82.55 0,0 97.79,0
Copper layers (1*16): Top 0.035mm / dielectric 1.5mm / Bottom 0.035mm
Design rules "default *": minimum track width 10mil, minimum drill 24mil, track to track 15mil, track to pad 15mil, pad to pad 15mil, via to via 15mil, smd to smd 8mil, copper to edge 40mil, drill to drill 8mil, minimum pad ring 10mil, minimum via ring 8mil, stop-mask expansion 4mil, vias tented up to drill 0mil, thermal gap 10mil

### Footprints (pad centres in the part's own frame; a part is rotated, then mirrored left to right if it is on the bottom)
2MMPINHDR_1X2 = drill 1.016 square: P$1 -1.49,0 | drill 1.016 octagon: P$2 0.51,0
SMT_CAP_2220 = smd 1.85 x 6.2: 1 -3,0; 2 3,0
C1206 = smd 1.6 x 1.8: 1 -1.4,0; 2 1.4,0
C0805 = smd 1.3 x 1.5: 1 -0.95,0; 2 0.95,0
C2220K = smd 1.85 x 5.5: 1 -2.55,0; 2 2.55,0
D/7343-31W = smd 2.95 x 2.7: + 3.375,0; - -3.375,0
R_1206 = smd 1.6 x 1.803: 1 -1.422,0; 2 1.422,0
2MMPINHDR_1X5 = drill 1.016 square: P$1 -0.22,0 | drill 1.016 octagon: P$2 1.78,0; P$3 3.78,0; P$4 5.78,0; P$5 7.78,0
1X11 = drill 1.016 pad 1.88: 1 0,0; 2 2.54,0; 3 5.08,0; 4 7.62,0; 5 10.16,0; 6 12.7,0; 7 15.24,0; 8 17.78,0; 9 20.32,0; 10 22.86,0; 11 25.4,0
1X05 = drill 1.016 long: 1 -5.08,0; 2 -2.54,0; 3 0,0; 4 2.54,0; 5 5.08,0
1X05' = drill 1.016 pad 1.88: 1 0,0; 2 2.54,0; 3 5.08,0; 4 7.62,0; 5 10.16,0
L1812 = smd 1.9 x 3.4: 1 -1.95,0; 2 1.95,0
1206 = smd 1.35 x 1.2: 1 -1.7,0; 2 1.65,0
L3225P = smd 1.8 x 2: 1 -1.4,0; 2 1.4,0
R0805 = smd 1.3 x 1.5: 1 -0.95,0; 2 0.95,0
R1210 = smd 1.6 x 2.7: 1 -1.4,0; 2 1.4,0
2MMPINHDR_1X1 = drill 1.016 square: P$1 0.034,0
DO-214AC(SMA) = smd 2.1 x 1.8: A -2.1,0; C 2.15,0
SO016 = smd 0.6 x 1.2: 1 -4.445,-2.8; 2 -3.175,-2.8; 3 -1.905,-2.8; 4 -0.635,-2.8; 5 0.635,-2.8; 6 1.905,-2.8; 7 3.175,-2.8; 8 4.445,-2.8; 9 4.445,2.8; 10 3.175,2.8; 11 1.905,2.8; 12 0.635,2.8; 13 -0.635,2.8; 14 -1.905,2.8; 15 -3.175,2.8; 16 -4.445,2.8
SOICW28_MICROCHIP = smd 0.65 x 1.7: 1 -7.62,-4.78; 2 -6.35,-4.78; 3 -5.08,-4.78; 4 -3.81,-4.78; 5 -2.54,-4.78; 6 -1.27,-4.78; 7 0,-4.78; 8 1.27,-4.78; 9 2.54,-4.78; 10 3.81,-4.78; 11 5.08,-4.78; 12 6.35,-4.78; 13 7.62,-4.78; 14 8.89,-4.78; 15 8.89,4.78; 16 7.62,4.78; 17 6.35,4.78; 18 5.08,4.78; 19 3.81,4.78; 20 2.54,4.78; 21 1.27,4.78; 22 0,4.78; 23 -1.27,4.78; 24 -2.54,4.78; 25 -3.81,4.78; 26 -5.08,4.78; 27 -6.35,4.78; 28 -7.62,4.78
SO8@1 = smd 0.6 x 2.2: 1 -1.905,-2.6; 2 -0.635,-2.6; 3 0.635,-2.6; 4 1.905,-2.6; 5 1.905,2.6; 6 0.635,2.6; 7 -0.635,2.6; 8 -1.905,2.6
DEUTSCH_EEC_325X-4B = drill 1.1 square: 1A 2.45,58.295; 1B 8.8,24.255 | drill 1.1: 2A 2.45,62.485; 2B 8.8,20.065; 3A 2.45,66.675; 3B 8.8,15.875; 4A 2.45,70.865; 4B 8.8,11.685; 5A 2.45,75.055; 5B 8.8,7.495; 6A 2.45,79.245; 6B 8.8,3.305; 7A 8.8,79.245; 7B 2.45,3.305; 8A 8.8,75.055; 8B 2.45,7.495; 9A 8.8,70.865; 9B 2.45,11.685; 10A 8.8,66.675; 10B 2.45,15.875; 11A 8.8,62.485; 11B 2.45,20.065; 12A 8.8,58.295; 12B 2.45,24.255 | hole 3.2: 4.41,41.28
SO8_GND_PAD = smd 0.6 x 2.2: 1 -2.032,-2.727; 2 -0.762,-2.727; 3 0.508,-2.727; 4 1.778,-2.727; 5 1.778,2.473; 6 0.508,2.473; 7 -0.762,2.473; 8 -2.032,2.473 | smd 6.35 x 1.905: 9 -0.127,0 | smd 7.62 x 5.08 bottom: 10 -0.127,-0.127 | drill 0.5: 11 -1.905,0; 12 -0.635,0; 13 0.635,0; 14 1.778,0
SO_08 = smd 0.6 x 2.2: 1 -1.905,-2.6; 2 -0.635,-2.6; 3 0.635,-2.6; 4 1.905,-2.6; 5 1.905,3.235; 6 0.635,3.235; 7 -0.635,3.235; 8 -1.905,3.235
FIDUCIAL_REV2 = smd 1 x 1: 1 0,0 | smd 1 x 1 bottom: 2 0,0
SO8 = smd 0.6 x 2.2: 1 -1.905,-2.6; 2 -0.635,-2.6; 3 0.635,-2.6; 4 1.905,-2.6; 5 1.905,2.6; 6 0.635,2.6; 7 -0.635,2.6; 8 -1.905,2.6
6-SMD_OMRON_SSRELAY = smd 1.5 x 2: 1 -3.81,-5.08; 2 -1.27,-5.08; 3 1.27,-5.08; 4 1.27,3.493; 5 -1.27,3.493; 6 -3.81,3.493
DPAK_TO263-3 = smd 1.27 x 2.997: 1 -2.553,-4.928; 2 -0.013,-4.928; 3 2.527,-4.928 | smd 12.7 x 7.62: 4 0,5.893

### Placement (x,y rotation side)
11V5_PWR  57.02,14.99 180 top
AUML1  17.27,29.97 270 top
BATT_PWR  5.71,28.45 270 top
C1  46.86,25.78 90 top
C2  93.85,15.88 270 top
C3  86.74,44.96 180 top
C4  31.75,63.25 0 top
C5  27.56,68.83 90 top
C6  82.17,45.59 180 top
C7  36.58,26.54 90 top
C8  88.9,53.47 270 top
C9  86.36,53.47 270 top
C10  68.96,72.01 90 top
C11  90.42,40.77 90 top
C12  77.09,45.59 180 top
C13  38.23,74.55 180 top
C14  42.8,30.86 180 top
C15  78.61,20.07 90 top
C16  15.49,44.58 180 top
C17  42.16,69.6 270 top
C18  64.52,11.05 270 top
C19  22.23,48.39 0 top
C20  29.46,45.09 270 top
C21  43.43,43.94 90 top
C22  90.68,16.13 270 top
C23  68.07,10.92 270 top
C24  35.31,58.55 0 top
C25  84.45,11.43 270 top
C26  84.2,72.9 90 top
C27  21.72,56.9 0 top
C28  40.26,49.78 180 top
C29  71.12,10.79 270 top
C30  65.02,61.47 180 top
C31  43.81,52.45 270 top
C32  21.84,51.69 0 top
C33  52.07,49.15 0 top
C34  50.29,25.53 90 top
C35  65.02,64.01 0 top
C36  90.3,35.81 270 top
C37  45.85,9.27 270 top
C38  56.77,7.24 90 top
C39  59.82,7.24 90 top
C40  53.85,62.23 0 top
C41  43.69,62.74 0 top
C42  43.69,60.07 0 top
C43  5.33,52.32 180 top
C44  5.21,48.9 180 top
C45  20.45,66.17 0 top
C46  57.53,73.53 90 top
C47  46.86,74.55 0 top
C48  46.86,77.22 0 top
C49  52.07,52.07 0 top
C51  90.3,31.88 180 top
F8  25.27,26.8 0 top
GND3  84.71,8.13 0 top
J4  80.14,54.61 180 top
JP1  66.04,34.29 180 top
JP2  82.17,49.15 180 top
JP3  breakout  [1X05']  95.12,43.56 270 top
L1  46.35,18.29 270 top
L2  50.93,18.29 270 top
L3  24.64,34.29 90 top
L4  29.72,34.29 90 top
L5  35.18,34.29 90 top
L6  41.91,18.29 270 top
L7  71.75,72.64 270 top
L8  76.07,73.41 270 top
L9  60.96,46.99 180 top
L10  60.58,42.29 90 top
L11  54.48,42.04 180 top
L12  62.74,51.05 90 top
L13  54.48,45.59 180 top
L14  59.31,51.05 90 top
P-UPS  69.09,61.98 270 top
R1  67.56,24.26 270 top
R2  64.26,26.16 270 top
R3  24.64,70.74 270 top
R4  20.83,69.72 180 top
R5  93.98,63.63 90 top
R6  68.45,16.89 270 top
R7  87.5,74.17 90 top
R8  90.04,74.17 90 top
R9  72.14,50.55 270 top
R11  15.24,61.59 180 top
R13  21.72,60.33 0 top
R14  21.84,54.23 180 top
R15  35.43,49.66 180 top
R16  28.32,53.21 90 top
R17  48.9,62.23 0 top
R18  64.52,16.89 270 top
R19  68.2,66.55 180 top
R20  68.58,58.8 180 top
R21  25.4,54.86 90 top
R22  38.23,71.37 0 top
R23  51.82,5.97 0 top
R24  52.07,10.41 0 top
R25  38.23,68.58 180 top
R26  15.24,76.45 180 top
R27  51.69,74.55 0 top
R28  24.64,66.17 270 top
R31  27.3,22.99 90 top
R32  26.16,13.21 90 top
TP1  31.5,76.83 0 top
TP2  43.81,56.26 90 top
TP3  15.75,48.01 270 top
TVS1  57.4,18.41 180 top
U1  82.93,38.86 180 top
U2  82.42,63.75 0 top
U3  22.35,43.94 90 top
U4  36.45,43.56 90 top
U5  15.24,55.24 180 top
U6  15.11,70.48 180 top
U$1  0,0 0 top
U$2  84.96,31.88 0 top
U$3  74.55,38.61 270 top
U$4  84.07,17.78 180 top
U$5  32.13,69.34 0 top
U$6  57.4,26.54 90 top
U$7  50.55,69.85 270 top
U$8  35.05,54.23 270 top
U$9  50.55,57.53 270 top
U$10  5.71,1.91 0 top
U$11  96.9,77.09 0 top
U$12  69.34,29.08 180 top
U$13  74.17,21.72 180 top
U$43  17.27,11.43 90 top
U$44  18.29,20.83 90 top
VREG3  34.8,14.35 180 top

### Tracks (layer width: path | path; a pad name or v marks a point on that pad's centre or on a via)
3V_AVDD
  Top 0.254: C10.1 L7.2
  Top 0.406: U2.28 72.72,69.93 L7.2
5V5  (via drill 0.5, 0.89)
  Top 0.813: U$6.1 64.32,18.48 R18.1 R6.1 v67.96,21.05 | R1.2 v67.96,21.05 | U$12.P$2 U$12.P$1 | v68.96,35.31 67.82,41.02 63.25,41.02 L10.1 | v67.96,21.05 67.96,20.32 68.12,20.16
  Bottom 0.813: 70.96,29.08 U$12.P$1 70.87,30.19 70.87,32.64 v68.96,35.31 | U$12.P$2 68.83,21.92 v67.96,21.05
5VF  (via drill 0.89)
  Top 0.61: U$4.8 86.11,13.02 C25.1 82.3,13.27 U$4.5
  Top 0.813: R6.2 R18.2 C18.1 | 70.99,11.87 C29.1 v71.12,13.34 | v81.03,12.7 81.73,12.7 82.3,13.27
  Top 1.27: C18.1 67.5,12.45 C23.1 70.99,11.87
  Bottom 0.813: v71.12,13.34 80.39,13.34 v81.03,12.7
  Bottom 1.27: v71.12,13.34 v71.12,8.26
11V5F  (via drill 0.51)
  Top 0.61: C38.1 | U$6.5 52.96,29.08 v50.16,29.08 | v50.16,22.86 50.81,24.06
  Top 0.813: 54.35,13.58 53.85,13.07 | 11V5_PWR.P$2 56.51,15.24 | TVS1.C 55.24,22.1 50.81,24.06 C34.1 | C34.1 47.06,24.58 C1.1 | U$6.8 50.36,24.51 C34.1
  Top 1.27: 53.85,13.07 R24.2 R23.2 53.85,5.84 C38.1 | 11V5_PWR.P$2 54.35,13.58 | 56.51,15.24 55.24,16.51 TVS1.C | C38.1 C39.1
  Bottom 0.61: v50.16,29.08 v50.16,22.86
12V  (via drill 0.89)
  Top 0.813: 50.29,5.84 R23.1
  Top 1.27: 32.26,19.79 VREG3.3 30.73,19.41 v30.73,19.3 | R24.1 R23.1 48.13,4.57 46.54,4.63 C37.+ 44.07,6.15 v43.18,9.53
  Bottom 1.27: v43.18,9.53 33.53,19.68 v30.73,19.3 27.94,20.68 25.02,22.1 22.07,20.04 18.09,20.04 U$1.2B
!CS1  (via drill 0.5)
  Top 0.406: U$9.7 55.75,58.17 v57.28,58.67 | v73.15,67.82 73.91,66.93 77.09,66.42 79.12,64.64 80.64,64.64 81.15,65.79 U2.23
  Bottom 0.406: v57.28,58.67 59.05,62.48 67.94,67.56 v73.15,67.82
!CS2  (via drill 0.51)
  Top 0.406: U$7.7 v56.13,70.48 | v63.75,70.48 64.64,71.37 64.64,78.23 v64.9,78.49 | v78.99,78.49 78.99,71.88 77.34,70.23 U2.26
  Bottom 0.406: v56.13,70.48 v63.75,70.48 | v64.9,78.49 v78.99,78.49
!MCLR
  Top 0.406: U2.1 74.72,58.97 72.39,56.64 72.39,54.64 J4.P$5 72.36,51.59 R9.1
A1
  Top 0.254: U5.7 15.88,54.86 18.92,54.86 R14.2
A2
  Top 0.406: U6.7 15.62,70.1 18.54,70.1 R4.2
AN1+
  Top 0.254: U5.4 11.68,60.2 10.54,64.14 5.08,64.77 U$1.3A
AN1-  (via drill 0.51)
  Top 0.254: U5.1 18.03,60.45 v18.03,63.25
  Bottom 0.254: v18.03,63.25 17.14,65.53 U$1.10A
AN2+
  Top 0.406: U6.4 11.43,73.08 11.43,76.96 4.83,76.96 4.83,79.25 U$1.6A
AN2-
  Top 0.406: U6.1 18.41,73.08 18.41,79.25 U$1.7A
AN_5V5  (via drill 0.51, 0.89)
  Top 0.406: C21.1 U4.2 U4.3 | v15.49,64.14 15.49,64.26 17.02,65.79 U6.8 C45.1 | U5.8 v18.67,51.56 C32.1
  Top 0.61: U$1.12A U$1.11A
  Top 0.813: L11.2 L13.2 | U$1.11A | C44.1 6.35,48.84 C43.1 U$1.12A | C21.1 v45.47,42.93 | 50.55,45.59 v50.15,46.2 50.67,46.2 C33.1 C49.1
  Top 1.27: v8.38,52.58 C43.1 | L13.2 50.55,45.59 50.42,45.59 v50.15,46.2
  Bottom 0.406: v15.49,64.14 11.94,64.9 U$1.11A | v18.67,51.56 14.22,53.85 v8.38,52.58
  Bottom 0.813: v45.47,42.93 v50.15,46.2
  Bottom 1.27: v45.47,42.93 41.53,40.26 10.92,40.26 8.51,47.62 v8.38,52.58
AN_GND  (via drill 0.5, 0.51, 0.9)
  Top 0.406: v43.43,46.74 C21.2 41.53,45.47 U4.4 | C20.2 v29.46,42.55 | C19.2 v24.89,47.24 U3.4 | C16.2 v13.46,42.8 | U5.5 v12.19,51.94 | C24.1 v32.51,58.8 | U$9.3 U$9.4 v46.86,54.48 | v40.51,62.87 C41.1 C42.1 | C28.1 v41.15,47.88 | U$8.4 v30.61,52.32 | R21.2 v25.4,57.91 | C32.2 v24.64,51.69 | C40.2 v56.52,62.99 | C4.1 v29.21,63.25 | U$5.4 v35.43,66.04 | U6.5 v11.81,68.2 | C45.2 23.24,65.28 R28.2 v22.99,65.28 | C13.1 39.18,75.12 v40.13,76.07 | C47.1 45.91,74.61 v44.7,75.82 45.91,77.03 C48.1 | U$7.4 U$7.3 47.95,67.12 v47.62,66.8 | C46.2 v57.53,76.2
  Top 0.813: L12.2 L14.2 | L14.2 v59.31,54.1 | C33.2 C49.2 v55.24,52.07 | L14.2
  Bottom 0.406: v46.86,54.48 46.23,54.23 | v40.51,62.87 54.74,67.82 | v41.15,47.88 40.26,47.24 | v30.61,52.32 29.84,52.32 | v25.4,57.91 24.64,58.93 | v24.64,51.69 25.15,50.67 | v56.52,62.99 56.77,63.88 | v29.21,63.25 28.07,63.25 | v35.43,66.04 35.56,64.9 | v11.81,68.2 10.79,68.83 | v22.99,65.28 22.73,64.52 | v40.13,76.07 40.13,76.71 40.26,76.83 | v44.7,75.82 44.2,75.82 44.07,75.69 | v47.62,66.8 47.24,66.8 46.86,66.42 | v57.53,76.2 57.53,76.58 57.28,76.83
  Bottom 0.813: 58.8,54.99 v59.31,54.1 59.31,52.07 v55.24,52.07
  pour Bottom: 0,40.64 60.96,40.64 60.96,83.82 0,83.82
ANI1
  Top 0.406: U$8.6 U$8.7 40.39,54.86 C31.1 TP2.P$1 46.48,58.17 U$9.2
ANI2  (via drill 0.51)
  Top 0.406: TP1.P$1 31.53,72.58 U$5.7 U$5.6 32.77,74.3 v33.66,75.18 | v42.04,72.14 42.04,70.67 C17.1 42.23,70.48 U$7.2
  Bottom 0.406: v33.66,75.18 37.47,75.18 40.51,72.14 v42.04,72.14
C1+
  Top 0.406: U1.1 87.38,43.31 87.76,43.69 87.76,45.53 C3.1
C1-
  Top 0.406: U1.3 84.84,43.31 85.6,44.07 85.6,45.4 C3.2
C2+
  Top 0.406: U1.4 83.57,43.81 83.19,44.2 83.19,45.53 C6.1
C2-
  Top 0.406: U1.5 82.3,42.93 81.28,43.94 81.28,45.53 C6.2
GND  (via drill 0.5, 0.6, 0.89, 0.9)  (2 unrouted)
  Top 0.254: C12.2 v74.42,44.7
  Top 0.406: C8.2 C9.2 86.55,52.52 v84.45,52.45 | U2.8 v83.69,61.47 | U2.19 v86.23,66.17 | C26.2 v84.07,75.69 | L8.1 74.22,75.11 v74.17,74.93 | C10.2 69.09,74.55 v68.96,74.68 | U1.15 v86.11,37.85 | C36.2 v88.9,33.53 89.35,32.7 C51.2 | C11.2 v91.06,43.31 | C14.2 JP1.11 | v63.75,59.56 C30.2 C35.1 | U$13.7 74.68,19.12 v74.68,21.46 73.91,22.23 73.53,22.23 U$13.3 U$13.4 | C15.2 v78.61,22.48 | C25.2 84.49,10.48 GND3.P$1
  Top 0.61: U$4.6 83.57,17.65 U$4.13 83.57,17.91 U$4.3 | C22.2 90.68,14.1 v91.69,13.08 93.09,14.47 C2.2 | U$44.2 v25.27,19.56 | U$43.2 v24.38,10.03
  Top 0.813: VREG3.4 v34.8,14.86 34.8,19.79 VREG3.2 | C1.2 46.99,27.3 48.77,27.3 49.6,26.48 C34.2 52.13,26.48 v52.7,27.05 U$6.6 | U$6.13 57.53,27.05 U$6.3 64.26,27.05 v64.26,28.96 64.2,27.62 R2.1 | 68.07,9.85 C23.2 | 64.71,9.46 C18.2 | L9.1 v63.12,45.59 | C43.2 3.93,49.73 C44.2 2.48,47.3 v1.91,43.43
  Top 1.27: L5.2 L4.2 L3.2 21.93,36.24 v21.84,36.2 | TVS1.A 59.5,15.98 11V5_PWR.P$1 | C29.2 68.07,9.85 | C23.2 64.71,9.46 | C18.2 v62.74,8.64 62.23,8.64 C39.2 C38.2 | C37.- 45.77,11.76 v48.01,13.08
  Bottom 0.254: v74.42,44.7 73.41,44.83
  Bottom 0.406: 88.77,32.64 88.9,32.51 | v83.69,61.47 83.69,62.23 83.82,62.36 | v86.23,66.17 86.23,65.41 86.36,65.28 | v84.07,75.69 84.2,75.56 | v74.17,74.93 74.42,74.8 73.91,74.8 | v68.96,74.68 68.96,75.18 69.22,75.44 | v86.11,37.85 86.11,38.48 | v88.9,33.53 88.9,33.4 90.42,33.02 | v91.06,43.31 91.31,43.31 91.57,43.56 | v63.75,59.56 63.75,59.31 | v74.68,21.46 74.04,21.46 74.04,21.59 | v78.61,22.48 78.61,22.86 78.87,22.86
  Bottom 0.61: v91.69,13.08 91.69,12.83 92.33,12.19 | v48.01,13.08 46.86,12.7 | v25.27,19.56 25.4,19.56 | v24.38,10.03 25.4,10.79
  Bottom 0.813: v34.8,14.86 34.67,14.86 34.67,16 | v21.84,36.2 21.97,36.2 | v52.7,27.05 52.2,27.05 51.94,26.8 | v64.26,28.96 64.26,28.7 | v1.91,43.43 1.91,43.56 1.52,37.85
  pour Bottom (no thermals): 0,-0.25 101.85,-0.25 101.85,82.68 62.23,82.68 62.48,38.61 -0.13,38.61
HV_PWM1
  Top 1.27: U$44.6 12.57,17.02 U$1.3B
HV_PWM2
  Top 1.27: U$43.6 12.06,7.62 U$1.4B
N$1
  Top 1.27: L2.1 L1.1 L6.1 41.91,21.84 39.89,23.87 C7.1 35.8,23.88 33.27,24 31.37,26.8 F8.2
N$2  (via drill 0.51)
  Top 0.254: R13.1 v20.7,62.23 | v29.34,60.45 36.32,60.45 C24.2
  Top 0.406: U$8.3 35.05,53.59 36.2,56.77 C24.2
  Bottom 0.254: v20.7,62.23 v29.34,60.45
N$3
  Top 0.813: VREG3.1 37.36,18.39 | 42.12,16.38 L6.2
  Top 1.27: 37.36,18.39 38.73,16.38 42.12,16.38 | L6.2 L1.2 L2.2
N$4  (via drill 0.5, 0.51)
  Top 0.254: C27.1 v19.3,58.29 | v28.07,56.26 R16.2
  Top 0.406: R16.2 30.35,54.86 U$8.2 U$8.1 v30.48,57.53
  Bottom 0.254: v19.3,58.29 24.77,55.63 26.54,55.63 v28.07,56.26
N$5
  Top 0.254: R14.1 C27.2 R13.2
  Top 0.406: R21.1 R14.1
N$6
  Top 0.813: R1.1 R2.2 64.2,25.27 62.61,25.27 62.1,25.78 U$6.2
N$7
  Top 0.813: L10.2 58.8,42.67 57.02,42.04 L11.1
  Top 1.27: L11.1 L13.1
N$8
  Top 0.406: U2.27 L8.2
N$9
  Top 0.406: C42.2 C41.2 R17.1 U$9.1
N$11  (via drill 0.89)
  other vias: 27.18,36.2
N$12  (via drill 0.89)
  other vias: 32.51,36.32
N$13  (via drill 0.5)
  Top 0.406: R15.2 v32.26,49.53 | v28.32,50.93 R16.1 | C31.2 v41.4,51.94
  Bottom 0.406: v28.32,50.93 v32.26,49.53 v41.4,51.94
N$14
  Top 0.406: R15.1 C28.2 U$8.5
N$15  (via drill 0.51)
  Top 0.406: C4.2 U$5.3 v32.77,68.96 | R3.1 v22.73,73.15
  Bottom 0.406: v22.73,73.15 v32.77,68.96
N$16
  Top 0.406: R4.1 R3.2 | R3.2 R28.1 | R3.2 C5.2
N$17
  Top 0.406: R22.2 R25.1 42.1,68.58 C17.2
N$18
  Top 0.406: U$5.5 34.99,72.58 36.2,71.37 R22.1 C13.2
N$19  (via drill 0.51)
  Top 0.406: U$5.2 U$5.1 | U$5.1 28.83,66.67 C5.1 | R25.2 v35.81,68.58 | v29.08,65.66 29.14,65.66 U$5.1
  Bottom 0.406: v35.81,68.58 35.31,68.58 32.38,65.66 v29.08,65.66
N$20
  Top 0.406: U$7.1 47.95,74.42 C47.2 | C47.2 R27.1 | C48.2 C47.2
N$22
  Top 0.61: R31.1 27.3,18.54 26.16,17.02 U$44.1
N$23
  Top 0.61: R32.1 26.16,7.62 U$43.1
PGC1
  Top 0.406: U2.5 79.88,56.64 80.26,56.26 80.26,54.7 J4.P$1
PGD1
  Top 0.406: U2.4 78.61,56.77 78.36,56.52 J4.P$2
PIC_RX1  (via drill 0.5)
  Top 0.254: U1.12 82.3,37.21 83.06,37.97 v83.82,37.97 | v93.98,60.96 R5.1 91.19,62.61 88.77,60.58 U2.12
  Top 0.406: 93.79,62.48 R5.1
  Bottom 0.254: v83.82,37.97 84.84,39.12 91.19,45.47 94.87,48.9 94.87,54.1 v93.98,60.96
PIC_RX2  (via drill 0.5)
  Top 0.254: U1.9 v78.49,37.34 | v91.44,57.02 U2.14
  Bottom 0.254: v91.44,57.02 92.17,50.47 92.2,50.16 82.3,39.5 v78.49,37.34 77.98,37.85 77.98,40.39 79.63,42.04 JP2.4
PIC_TX1  (via drill 0.5)
  Top 0.254: U1.11 81.03,37.34 v81.79,38.1 | v87.5,61.34 U2.11
  Bottom 0.254: v81.79,38.1 83.19,39.24 86.23,42.16 93.85,49.78 93.6,56.39 92.96,58.8 90.42,60.83 v87.5,61.34
PIC_TX2  (via drill 0.5)
  Top 0.254: U2.10 v86.23,57.15 | v79.76,39.24 U1.10
  Bottom 0.254: v86.23,57.15 90.3,56.01 90.3,50.42 81.92,40.26 v79.76,39.24 79.5,39.5 79.5,40.26 82.17,42.93 JP2.3
PWM1  (via drill 0.51, 0.89)
  Top 0.406: U2.15 v92.84,68.71 | v89.15,64.52 83.06,64.26 v79.76,61.59 | v70.48,55.88 v69.47,53.09
  Top 0.61: v29.97,24.51 R31.2
  Bottom 0.406: v29.97,24.51 38.35,37.21 66.17,37.21 69.47,39.75 v69.47,53.09 | v92.84,68.71 v89.15,64.52 | v79.76,61.59 75.69,57.28 v70.48,55.88
PWM2  (via drill 0.51)
  Top 0.406: U2.16 90.04,70.23 91.19,71.37 92.96,71.37 v93.22,71.12 | v88.52,63.12 83.31,63.12 v81.41,61.59 | v75.82,52.45 74.42,49.15 v74.17,47.12 | v31.75,22.61 29.34,20.83 28.7,20.19 28.7,18.03
  Top 0.61: 28.7,18.03 R32.2
  Bottom 0.406: v93.22,71.12 93.22,70.99 94.74,69.47 94.74,67.82 94.49,67.82 89.92,63.25 88.65,63.25 v88.52,63.12 | v81.41,61.59 81.41,61.21 82.42,56.26 82.42,54.36 81.28,52.45 v75.82,52.45 | v74.17,47.12 70.87,45.59 70.87,38.99 67.18,36.32 38.99,36.2 32.13,23.75 31.88,23.24 v31.75,22.61
PWR_GND  (via drill 0.89)
  Top 0.813: 17.57,32.89 AUML1.1 | 29.97,32.09 L4.1 | L3.1 23.58,32.34 23.37,32.13
  Top 1.27: 12.32,32.89 11.94,32.89 9.74,29.94 BATT_PWR.P$1 4.19,29.97 2.41,28.96 U$1.12B | 12.32,32.89 17.57,32.89 20.7,32.89 21.46,32.13 23.37,32.13 | C7.2 32.89,29.09 29.97,32.09 | L3.1 L4.1 L5.1 | v12.32,30.99 12.32,32.89 | U$44.4 18.67,22.1 v18.67,23.5 18.67,12.7 U$43.4
  Bottom 1.27: v18.67,23.5 v12.32,30.99
PWR_GND1
  Top 0.813: L9.2 59.18,49.66 L12.1 L14.1
RG+_0
  Top 0.406: U5.2 15.88,59.56 16.13,60.45 R11.1
RG+_1
  Top 0.406: U6.2 15.75,74.8 15.88,74.8 15.88,75.95 16.06,76.2 R26.1
RG-_0
  Top 0.406: U5.3 14.61,59.44 14.22,60.45 R11.2
RG-_1
  Top 0.406: U6.3 14.48,74.8 14.29,74.8 R26.2
RS_RX1  (via drill 0.5)
  Top 0.254: v91.06,28.07 v91.06,24
  Top 0.406: U1.13 83.57,33.66 83.44,33.53 83.44,31.91 U$2.P$1
  Bottom 0.254: 83.82,30.23 v91.06,28.07 | v91.06,24 92.71,24.38 96.9,23.5 99.57,20.7 99.57,5.33 94.36,1.91 10.92,1.91 8.38,1.27 6.48,2.29 4.19,3.3 U$1.7B
  Bottom 0.406: 83.82,30.23 U$2.P$1
RS_RX2  (via drill 0.5)
  Top 0.254: U$3.P$1 73.03,38.86 73.03,37.21 74.04,36.45 75.31,35.69 76.33,34.42 v78.74,32.38 | v86.11,27.3 v86.11,23.62
  Top 0.406: U1.8 76.11,41.66 U$3.P$1
  Bottom 0.254: v78.74,32.38 79.63,30.86 80.52,29.84 82.42,28.32 v86.11,27.3 | v86.11,23.62 87.76,21.84 94.87,18.41 94.87,7.62 93.22,6.35 42.42,5.84 26.42,5.71 11.81,6.48 10.41,9.4 6.22,9.4 3.94,7.49 U$1.8B
RS_TX1  (via drill 0.5)
  Top 0.254: v92.58,28.57 v92.58,22.73
  Top 0.406: U1.14 84.84,34.16 85.47,33.53 U$2.P$2
  Bottom 0.254: v92.58,22.73 96.14,22.23 98.3,19.56 98.3,6.1 93.98,3.3 U$1.6B
  Bottom 0.406: v92.58,28.57 91.19,29.59 U$2.P$2
RS_TX2  (via drill 0.5)
  Top 0.254: U1.7 79.76,40.51 76.83,40.01 76.83,38.1 U$3.P$2 | U$3.P$2 76.33,35.81 77.22,34.92 v80.14,33.02 | v89.03,27.56 v89.03,23.5
  Top 0.406: U$3.P$2
  Bottom 0.254: v80.14,33.02 82.8,29.08 v89.03,27.56 | v89.03,23.5 91.57,21.46 96.52,18.92 96.65,6.73 93.6,4.83 11.18,4.57 U$1.5B
RST  (via drill 0.5)
  Top 0.254: v83.95,56.64 84.96,57.66 U2.9
  Bottom 0.254: JP2.5 77.09,51.18 77.22,51.44 81.79,51.44 83.95,54.99 v83.95,56.64
SCK1  (via drill 0.5, 0.51)
  Top 0.406: U$9.5 v56.13,55.63 | v78.61,66.67 U2.25 | U$7.5 v55.63,66.93 | v58.8,64.26 v60.02,61.29
  Bottom 0.406: v56.13,55.63 57.28,55.63 58.42,57.4 59.73,60.59 v60.02,61.29 60.2,61.72 67.56,66.29 v78.61,66.67 | v55.63,66.93 v58.8,64.26
SCL1  (via drill 0.5)
  Top 0.406: U2.17 88.77,70.99 90.3,72.64 R8.1 90.68,73.15 94.36,73.15 98.68,67.18 98.68,41.02 | JP1.8 48.26,32.38 74.04,32.38 79.48,28.04 | 79.48,28.04 79.76,27.81 v79.88,27.74 | v79.88,27.74 v82.42,26.29 | v94.61,26.29 98.68,26.29 98.68,41.02 | U$13.1 76.77,24.32 v77.34,24.89 | v79.88,27.74 79.77,27.74 79.48,28.04 | JP3.2 98.68,41.02
  Bottom 0.406: v82.42,26.29 v94.61,26.29 | v77.34,24.89 77.34,25.21 v79.88,27.74
SDA1  (via drill 0.5)
  Top 0.406: R7.1 U2.18 87.5,67.31 88.14,66.67 96.39,66.67 96.39,57.28 arc-90 v97.41,57.02 | v68.2,31.37 72.26,31.11 74.66,30.33 | 74.66,30.33 v75.03,30.04 | v75.03,30.04 78.36,27.43 v81.15,25.15 | U$13.2 v74.8,26.67 | v75.03,30.04 74.95,30.04 74.66,30.33
  Bottom 0.406: JP1.9 45.72,31.37 v68.2,31.37 | v81.15,25.15 97.54,25.15 97.48,38.61 | 97.48,38.61 v97.41,57.02 | v74.8,26.67 74.8,29.82 v75.03,30.04 | JP3.3 97.35,38.48 97.48,38.61
SDI1  (via drill 0.5)
  Top 0.254: U2.22 82.42,70.1 81.41,71.12 81.41,76.58 v81.28,76.71 | U$7.6 v51.18,69.22 v51.18,65.28 | U$9.6 51.31,56.9 v51.18,57.02
  Bottom 0.254: v81.28,76.71 60.2,76.71 58.55,78.36 54.23,78.36 51.05,75.18 51.05,69.34 v51.18,69.22 | v51.18,57.02 v51.18,65.28
SW1  (via drill 0.5, 0.6)
  Top 0.406: C35.2 66.01,63.47 P-UPS.P$1 69.09,66.49 R19.1 | U2.2 76.07,60.58 v74.17,62.48 70.87,57.28 67.82,56.01 v67.82,53.72 | v9.65,34.54 15.75,38.48 37.21,38.48 45.85,38.23 63.75,38.23 v65.91,39.12
  Bottom 0.254: v74.17,62.48 71.25,63.37 P-UPS.P$1
  Bottom 0.406: 69.12,63.5 P-UPS.P$1 | v9.65,34.54 8.38,27.05 6.48,25.15 6.48,19.9 U$1.10B | v65.91,39.12 67.94,40.39 v67.82,53.72
SW2  (via drill 0.5, 0.6)
  Top 0.406: v77.34,61.85 U2.3 | v6.6,34.29 15.75,39.62 37.21,39.62 45.72,38.99 61.34,38.99 v64.26,39.62 | v65.15,57.4 C30.1 66.1,60.96 67.56,60.96 68.07,61.47 P-UPS.P$2 69.6,60.26 R20.1
  Bottom 0.254: 74.55,60.83 P-UPS.P$2
  Bottom 0.406: v77.34,61.85 76.45,61.85 74.55,60.83 | P-UPS.P$2 | v6.6,34.29 5.33,34.29 2.92,30.61 3.17,26.92 5.08,25.02 5.08,22.7 U$1.11B | v64.26,39.62 66.55,41.53 v65.15,57.4
V+
  Top 0.406: U1.2 86.11,40.64 86.87,39.88 91,39.88 C11.1
V-
  Top 0.406: U1.6 81.03,42.61 C12.1
VBATT
  Top 0.813: 17.22,26.92 AUML1.2 | 23.68,26.97 F8.1
  Top 1.27: 17.22,26.92 11.94,26.92 10.92,27.94 BATT_PWR.P$2 U$1.1B | AUML1.2 23.68,26.97
VCAP
  Top 0.406: U2.20 84.96,69.72 C26.1
VCC
  Top 0.406: C14.1 JP1.10
  Top 0.61: U$4.2 U$4.1 88.08,20.57 C22.1 93.66,17.08 C2.1 | JP1.10 43.69,31.37 63.25,31.37
  pour Top: 62.61,-0.25 101.6,0 101.6,83.82 62.61,83.57
VREF_2V5  (via drill 0.51)
  Top 0.406: U3.6 C16.1 TP3.P$1 14.61,50.42 U5.6 14.61,54.86 v11.56,56.13 | v12.32,63.25 14.48,65.28 U6.6
  Bottom 0.406: v11.56,56.13 11.56,61.59 v12.32,63.25
VREF_3V3
  pour Top: 0,40.64 60.96,40.64 60.96,83.82 0,83.82

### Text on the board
tPlace: DH_HV_precAn_6_6_14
